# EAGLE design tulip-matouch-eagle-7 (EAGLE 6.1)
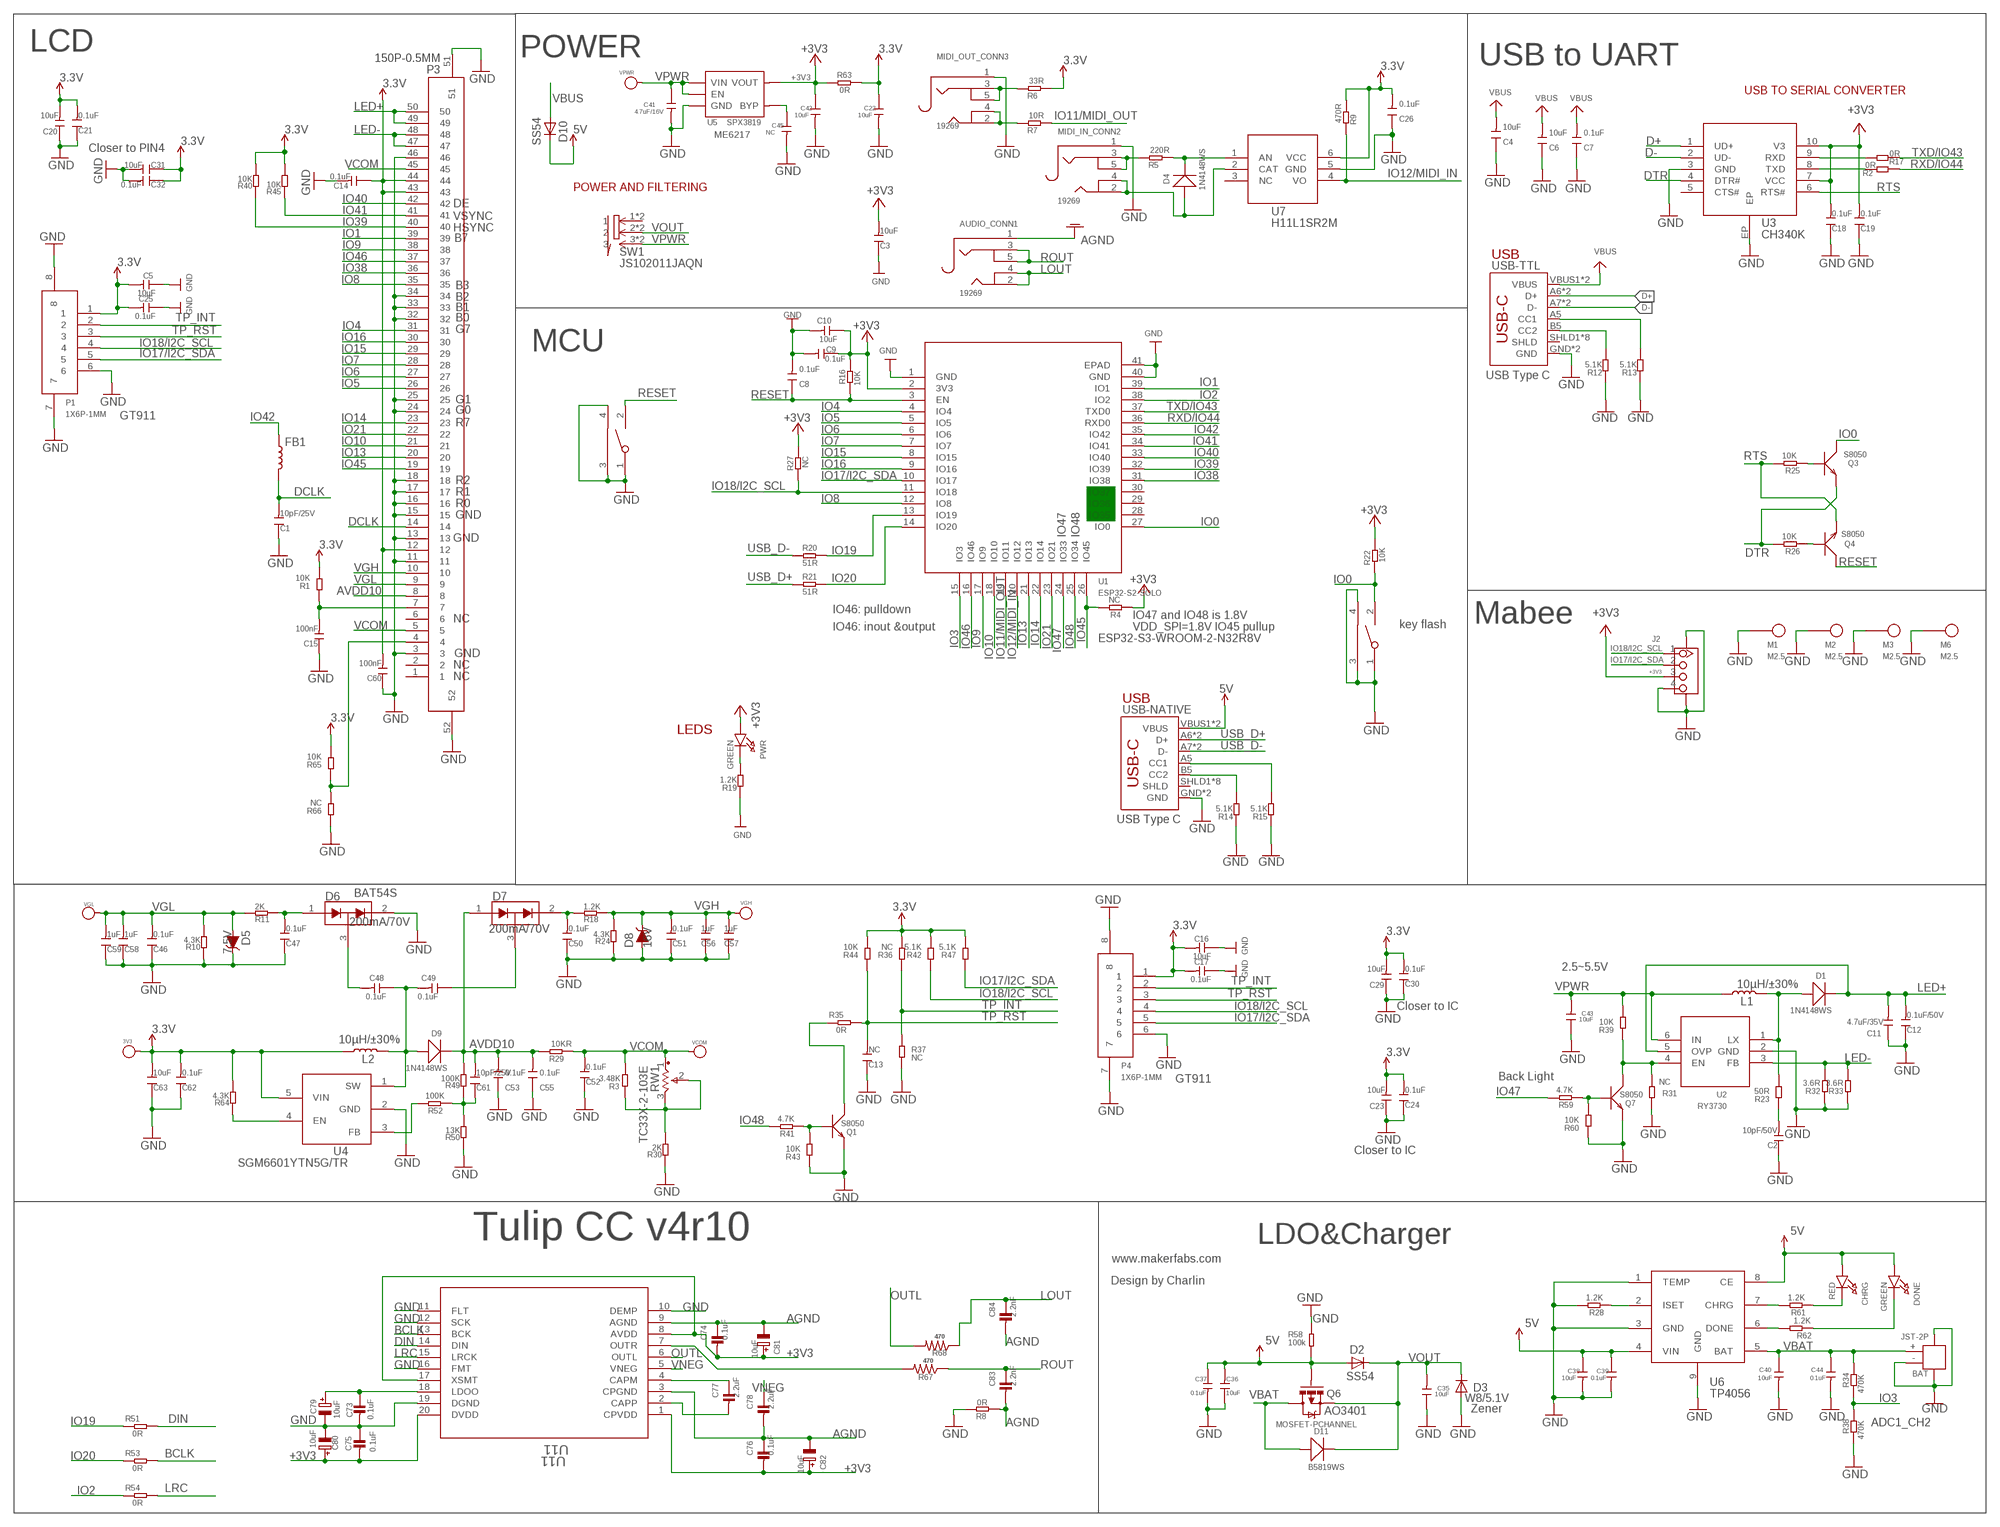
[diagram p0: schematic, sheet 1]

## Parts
3V3  PAD-TEST-POINT-CIRCLE'4545'  [TP_4545]
AUDIO_CONN1  19269  AUDIO_3.5MMJACK  [4UCONN_19269]
BAT  JST-2P  JST-2P-SMD'2.0'  [HW2-SMD-2.0-90D]
BOOT  TS24CA  [2*4*3.5MM]
C1  10pF/25V  DISCRETE_C-0603  [DISCRETE_C0603]
C2  10pF/50V  DISCRETE_C-0603  [DISCRETE_C0603]
C3  10uF  DISCRETE_C-0603  [DISCRETE_C0603]
C4  10uF  DISCRETE_C-0603  [DISCRETE_C0603]
C5  10uF  DISCRETE_C-0603  [DISCRETE_C0603]
C6  10uF  DISCRETE_C-0603  [DISCRETE_C0603]
C7  0.1uF  DISCRETE_C-0603  [DISCRETE_C0603]
C8  0.1uF  DISCRETE_C-0603  [DISCRETE_C0603]
C9  0.1uF  DISCRETE_C-0603  [DISCRETE_C0603]
C10  10uF  DISCRETE_C-0603  [DISCRETE_C0603]
C11  4.7uF/35V  DISCRETE_C-1206  [DISCRETE_C1206]
C12  0.1uF/50V  DISCRETE_C-0603  [DISCRETE_C0603]
C13  NC  DISCRETE_C-0603  [DISCRETE_C0603]
C14  0.1uF  DISCRETE_C-0603  [DISCRETE_C0603]
C15  100nF  DISCRETE_C-0603  [DISCRETE_C0603]
C16  10uF  DISCRETE_C-0603  [DISCRETE_C0603]
C17  0.1uF  DISCRETE_C-0603  [DISCRETE_C0603]
C18  0.1uF  DISCRETE_C-0603  [DISCRETE_C0603]
C19  0.1uF  DISCRETE_C-0603  [DISCRETE_C0603]
C20  10uF  DISCRETE_C-0603  [DISCRETE_C0603]
C21  0.1uF  DISCRETE_C-0603  [DISCRETE_C0603]
C22  10uF  C-0603  [0603]
C23  10uF  DISCRETE_C-0603  [DISCRETE_C0603]
C24  0.1uF  DISCRETE_C-0603  [DISCRETE_C0603]
C25  0.1uF  DISCRETE_C-0603  [DISCRETE_C0603]
C26  0.1uF  DISCRETE_C-0603  [DISCRETE_C0603]
C29  10uF  DISCRETE_C-0603  [DISCRETE_C0603]
C30  0.1uF  DISCRETE_C-0603  [DISCRETE_C0603]
C31  10uF  DISCRETE_C-0603  [DISCRETE_C0603]
C32  0.1uF  DISCRETE_C-0603  [DISCRETE_C0603]
C35  10uF  C-0603  [0603]
C36  10uF  C-0603  [0603]
C37  0.1uF  C-0603  [0603]
C38  10uF  C-0603  [0603]
C39  0.1uF  C-0603  [0603]
C40  10uF  C-0603  [0603]
C41  4.7uF/16V  C-0603  [0603]
C42  10uF  C-0603  [0603]
C43  10uF  C-0603  [0603]
C44  0.1uF  C-0603  [0603]
C45  NC  C-0603  [0603]
C46  0.1uF  DISCRETE_C-0603  [DISCRETE_C0603]
C47  0.1uF  DISCRETE_C-0603  [DISCRETE_C0603]
C48  0.1uF  DISCRETE_C-0603  [DISCRETE_C0603]
C49  0.1uF  DISCRETE_C-0603  [DISCRETE_C0603]
C50  0.1uF  DISCRETE_C-0603  [DISCRETE_C0603]
C51  0.1uF  DISCRETE_C-0603  [DISCRETE_C0603]
C52  0.1uF  DISCRETE_C-0603  [DISCRETE_C0603]
C53  0.1uF  DISCRETE_C-0603  [DISCRETE_C0603]
C55  0.1uF  DISCRETE_C-0603  [DISCRETE_C0603]
C56  1uF  DISCRETE_C-0603  [DISCRETE_C0603]
C57  1uF  DISCRETE_C-0603  [DISCRETE_C0603]
C58  1uF  DISCRETE_C-0603  [DISCRETE_C0603]
C59  1uF  DISCRETE_C-0603  [DISCRETE_C0603]
C60  100nF  DISCRETE_C-0603  [DISCRETE_C0603]
C61  10pF/25V  DISCRETE_C-0603  [DISCRETE_C0603]
C62  0.1uF  DISCRETE_C-0603  [DISCRETE_C0603]
C63  10uF  DISCRETE_C-0603  [DISCRETE_C0603]
C73  0.1uF  CAP_CERAMIC0805-NOOUTLINE  [0805-NO]
C74  0.1uF  CAP_CERAMIC0805-NOOUTLINE  [0805-NO]
C75  0.1uF  CAP_CERAMIC0805-NOOUTLINE  [0805-NO]
C76  0.1uF  CAP_CERAMIC0805-NOOUTLINE  [0805-NO]
C77  2.2uF  CAP_CERAMIC0805-NOOUTLINE  [0805-NO]
C78  2.2uF  CAP_CERAMIC0805-NOOUTLINE  [0805-NO]
C79  10uF  CAP_ELECTROLYTICPANASONIC_C  [PANASONIC_C]
C80  10uF  CAP_ELECTROLYTICPANASONIC_C  [PANASONIC_C]
C81  10uF  CAP_ELECTROLYTICPANASONIC_C  [PANASONIC_C]
C82  10uF  CAP_ELECTROLYTICPANASONIC_C  [PANASONIC_C]
C83  2.2nF  CAP_CERAMIC0805-NOOUTLINE  [0805-NO]
C84  2.2nF  CAP_CERAMIC0805-NOOUTLINE  [0805-NO]
CHRG  RED  LED0805_NOOUTLINE  [CHIPLED_0805_NOOUTLINE]
D1  1N4148WS  D'0805'  [SOD323]
D2  SS54  DIODE-DO-214AC  [DO-214AC]
D3  W8/5.1V  DIODE-SOD123  [SOD123]
D4  1N4148WS  D'0805'  [SOD323]
D5  7.5V  DIODE-ZENER-MMSZ5232BS  [SOD-323]
D6  200mA/70V  BAV99  [SOT23-3]
D7  200mA/70V  BAV99  [SOT23-3]
D8  16V  DIODE-ZENER-MMSZ5232BS  [SOD-323]
D9  1N4148WS  D'0805'  [SOD323]
D10  SS54  DIODE-DO-214AC  [DO-214AC]
D11  B5819WS  D'0805'  [SOD323]
DONE  GREEN  LED0805_NOOUTLINE  [CHIPLED_0805_NOOUTLINE]
FB1  INDUCTORFB-30OHM  [0603]
J2  GROVE-CONNECTOR-SMD'90D'  [HW4-SMD-2.0-90D]
L1  10µH/±30%  INDUCTOR-CR54-3.3UH  [CR54]
L2  10µH/±30%  INDUCTOR-CR54-3.3UH  [CR54]
M1  M2.5  [M2.5]
M2  M2.5  [M2.5]
M3  M2.5  [M2.5]
M6  M2.5  [M2.5]
MIDI_IN_CONN2  19269  AUDIO_3.5MMJACK  [4UCONN_19269]
MIDI_OUT_CONN3  19269  AUDIO_3.5MMJACK  [4UCONN_19269]
P1  1X6P-1MM  [1*6P-SMT1MM]
P3  150P-0.5MM  [1*50P-SMT0.5MM]
P4  1X6P-1MM  [1*6P-SMT1MM]
PWR  GREEN  LED0805_NOOUTLINE  [CHIPLED_0805_NOOUTLINE]
Q1  S8050  TRANSISTOR-NPN-SOT23  [SOT23]
Q3  S8050  TRANSISTOR-NPN-SOT23  [SOT23]
Q4  S8050  TRANSISTOR-NPN-SOT23  [SOT23]
Q6  MOSFET-PCHANNEL  [SOT23-3]
Q7  S8050  TRANSISTOR-NPN-SOT23  [SOT23]
R1  10K  DISCRETE_R-0603  [DISCRETE_R0603]
R2  0R  R-0603  [R0603]
R3  3.48K  DISCRETE_R-0603  [DISCRETE_R0603]
R4  NC  R-0603  [R0603]
R5  220R  R-0603  [R0603]
R6  33R  R-0603  [R0603]
R7  10R  R-0603  [R0603]
R8  0R  DISCRETE_R-0603  [DISCRETE_R0603]
R9  470R  R-0603  [R0603]
R10  4.3K  DISCRETE_R-0603  [DISCRETE_R0603]
R11  2K  DISCRETE_R-0603  [DISCRETE_R0603]
R12  5.1K  DISCRETE_R-0603  [DISCRETE_R0603]
R13  5.1K  DISCRETE_R-0603  [DISCRETE_R0603]
R14  5.1K  DISCRETE_R-0603  [DISCRETE_R0603]
R15  5.1K  DISCRETE_R-0603  [DISCRETE_R0603]
R16  10K  R-0603  [R0603]
R17  0R  R-0603  [R0603]
R18  1.2K  DISCRETE_R-0603  [DISCRETE_R0603]
R19  1.2K  DISCRETE_R-0603  [DISCRETE_R0603]
R20  51R  R-0603  [R0603]
R21  51R  R-0603  [R0603]
R22  10K  R-0603  [R0603]
R23  50R  DISCRETE_R-0603  [DISCRETE_R0603]
R24  4.3K  DISCRETE_R-0603  [DISCRETE_R0603]
R25  10K  R-0603  [R0603]
R26  10K  R-0603  [R0603]
R27  NC  R-0603  [R0603]
R28  1.2K  R-0603  [R0603]
R29  10KR  DISCRETE_R-0603  [DISCRETE_R0603]
R30  2K  DISCRETE_R-0603  [DISCRETE_R0603]
R31  NC  DISCRETE_R-0603  [DISCRETE_R0603]
R32  3.6R  DISCRETE_R-0603  [DISCRETE_R0603]
R33  3.6R  DISCRETE_R-0603  [DISCRETE_R0603]
R34  470K  R-0603  [R0603]
R35  0R  R-0603  [R0603]
R36  NC  DISCRETE_R-0603  [DISCRETE_R0603]
R37  NC  DISCRETE_R-0603  [DISCRETE_R0603]
R38  470K  R-0603  [R0603]
R39  10K  DISCRETE_R-0603  [DISCRETE_R0603]
R40  10K  DISCRETE_R-0603  [DISCRETE_R0603]
R41  4.7K  DISCRETE_R-0603  [DISCRETE_R0603]
R42  5.1K  DISCRETE_R-0603  [DISCRETE_R0603]
R43  10K  DISCRETE_R-0603  [DISCRETE_R0603]
R44  10K  DISCRETE_R-0603  [DISCRETE_R0603]
R45  10K  DISCRETE_R-0603  [DISCRETE_R0603]
R47  5.1K  DISCRETE_R-0603  [DISCRETE_R0603]
R49  100K  DISCRETE_R-0603  [DISCRETE_R0603]
R50  13K  DISCRETE_R-0603  [DISCRETE_R0603]
R51  0R  R-0603  [R0603]
R52  100K  DISCRETE_R-0603  [DISCRETE_R0603]
R53  0R  R-0603  [R0603]
R54  0R  R-0603  [R0603]
R58  100k  R-0603  [R0603]
R59  4.7K  DISCRETE_R-0603  [DISCRETE_R0603]
R60  10K  DISCRETE_R-0603  [DISCRETE_R0603]
R61  1.2K  R-0603  [R0603]
R62  1.2K  R-0603  [R0603]
R63  0R  R-0603  [R0603]
R64  4.3K  DISCRETE_R-0603  [DISCRETE_R0603]
R65  10K  DISCRETE_R-0603  [DISCRETE_R0603]
R66  NC  DISCRETE_R-0603  [DISCRETE_R0603]
R67  470  R-US_R0805  [R0805]
R68  470  R-US_R0805  [R0805]
RST  TS24CA  [2*4*3.5MM]
RW1  TC33X-2-103E  [TC33-3MM-SMD]
SW1  JS102011JAQN  [SMD-6-2.5MM]
U1  ESP32­S2­SOLO  [ESP32-­S2-­SOLO]
U2  RY3730  [SOT23-6]
U3  CH340K  [ESOP-10-EP-150MIL]
U4  SGM6601YTN5G/TR  [SOT-23-5]
U5  SPX3819  [SOT23-5]
U6  TP4056  [SOP8-1.27P]
U7  H11L1SR2M  [SOP-6-2.54MM]
U11  U11  PCM5101APW  [PW20_TEX]
USB-NATIVE  USB_C5  [USB-C-16P-5]
USB-TTL  USB_C5  [USB-C-16P-5]
VCOM  PAD-TEST-POINT-CIRCLE'4545'  [TP_4545]
VGH  PAD-TEST-POINT-CIRCLE'4545'  [TP_4545]
VGL  PAD-TEST-POINT-CIRCLE'4545'  [TP_4545]
VPWR  PAD-TEST-POINT-CIRCLE'4545'  [TP_4545]

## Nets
3.3V: 3V3.T C5.2 C14.1 C16.2 C17.2 C20.2 C21.2 C22.1 C23.2 C24.2 C25.2 C26.2 C29.2 C30.2 C31.1 C32.1 C60.2 C62.2 C63.2 L2.P$1 P1.1 P3.12 P3.43 P3.44 P4.1 R1.2 R6.1 R9.1 R36.2 R40.2 R42.2 R44.2 R45.2 R47.2 R63.2 R64.2 R65.2 U4.5(VIN) U7.6(VCC)
5V: C36.2 C37.1 C38.1 C39.1 CHRG.A D2.A D10.C DONE.A Q6.1(G) R58.1 U6.4(VIN) U6.8(CE) USB-NATIVE.VBUS1(VBUS) USB-NATIVE.VBUS2(VBUS)
+3V3: C3.2 C9.1 C10.1 C18.2 C19.2 C42.1 C74.2 C75.2 C76.2 C80.+ C81.+ C82.+ J2.3 PWR.A R4.1 R16.2 R22.2 R27.2 R63.1 U1.2(3V3) U3.7(VCC) U3.10(V3) U5.5(VOUT) U11.1(CPVDD) U11.8(AVDD) U11.17(XSMT) U11.20(DVDD)
AGND: AUDIO_CONN1.1 C74.1 C76.1 C78.2 C81.- C82.- C83.2 C84.2 R8.1 U11.3(CPGND) U11.9(AGND)
AVDD10: C53.2 C55.2 C61.2 D7.1(A1) D9.- P3.8 R29.2 R49.2
BCLK: R53.2 U11.13(BCK)
D+: U3.1(UD+) USB-TTL.A6(D+) USB-TTL.B6(D+)
D-: U3.2(UD-) USB-TTL.A7(D-) USB-TTL.B7(D-)
DCLK: C1.2 FB1.2 P3.14
DIN: R51.2 U11.14(DIN)
DTR: Q3.2(E) R26.2 U3.4(DTR#)
GND: BAT.3 BAT.4 BAT.- BOOT.1 BOOT.3 BOOT.4 C1.1 C2.1 C3.1 C4.1 C5.1 C6.1 C7.1 C8.2 C9.2 C10.2 C11.1 C12.1 C13.1 C14.2 C15.1 C16.1 C17.1 C18.1 C19.1 C20.1 C21.1 C22.2 C23.1 C24.1 C25.1 C26.1 C29.1 C30.1 C31.2 C32.2 C35.1 C36.1 C37.2 C38.2 C39.2 C40.2 C41.2 C42.2 C43.1 C44.2 C45.2 C46.1 C47.1 C50.1 C51.1 C52.1 C53.1 C55.1 C56.1 C57.1 C58.1 C59.1 C60.1 C62.1 C63.1 C73.2 C75.1 C79.- C80.- D3.A D5.C D6.2(C2) D8.A J2.4 J2.SS1 J2.SS2 M1.1 M2.1 M3.1 M6.1 MIDI_IN_CONN2.1 MIDI_OUT_CONN3.1 P1.6 P1.7 P1.8 P3.3 P3.11 P3.13 P3.15 P3.16 P3.17 P3.18 P3.24 P3.25 P3.32 P3.33 P3.34 P3.46 P3.51 P3.52 P4.6 P4.7 P4.8 Q1.2(E) Q7.2(E) R8.2 R10.1 R12.1 R13.1 R14.1 R15.1 R19.1 R24.1 R28.2 R30.1 R31.1 R32.1 R33.1 R37.2 R38.1 R43.1 R50.1 R58.2 R60.1 R66.1 RST.1 RST.3 RST.4 U1.1(GND) U1.40(GND) U1.41(EPAD) U2.2(GND) U3.3(GND) U3.EP U4.2(GND) U5.2(GND) U6.1(TEMP) U6.3(GND) U6.9(GND) U7.5(GND) U11.10(DEMP) U11.11(FLT) U11.12(SCK) U11.16(FMT) U11.19(DGND) USB-NATIVE.GND USB-NATIVE.GND2(GND) USB-TTL.GND USB-TTL.GND2(GND)
IO0: BOOT.2 Q3.3(C) R22.1 U1.27(IO0)
IO1: P3.39 U1.39(IO1)
IO2: R54.1 U1.38(IO2)
IO3: R34.1 R38.2 U1.15(IO3)
IO4: P3.31 U1.4(IO4)
IO5: P3.26 U1.5(IO5)
IO6: P3.27 U1.6(IO6)
IO7: P3.28 U1.7(IO7)
IO8: P3.35 U1.12(IO8)
IO9: P3.38 U1.17(IO9)
IO10: P3.21 U1.18(IO10)
IO11/MIDI_OUT: R7.1 U1.19(IO11)
IO12/MIDI_IN: R9.2 U1.20(IO12) U7.4(VO)
IO13: P3.20 U1.21(IO13)
IO14: P3.23 U1.22(IO14)
IO15: P3.29 U1.8(IO15)
IO16: P3.30 U1.9(IO16)
IO17/I2C_SDA: J2.2 P1.5 P4.5 R47.1 U1.10(IO17)
IO18/I2C_SCL: J2.1 P1.4 P4.4 R27.1 R42.1 U1.11(IO18)
IO19: R20.2 R51.1 U1.13(IO19)
IO20: R21.2 R53.1 U1.14(IO20)
IO21: P3.22 U1.23(IO21)
IO38: P3.36 U1.31(IO38)
IO39: P3.40 R40.1 U1.32(IO39)
IO40: P3.42 U1.33(IO40)
IO41: P3.41 R45.1 U1.34(IO41)
IO42: FB1.1 U1.35(IO42)
IO45: P3.19 R4.2 U1.26(IO45)
IO46: P3.37 U1.16(IO46)
IO47: R59.2 U1.24(IO33)
IO48: R41.2 U1.25(IO34)
LCD_RST: C15.2 P3.7 R1.1
LED+: C11.2 C12.2 D1.- P3.49 P3.50 U2.5(OVP)
LED-: P3.47 P3.48 R32.2 R33.2 U2.3(FB)
LOUT: AUDIO_CONN1.2 AUDIO_CONN1.4 C84.1 R68.1
LRC: R54.2 U11.15(LRCK)
N$1: C47.2 D6.1(A1) R11.1
N$2: Q4.1(B) R26.1
N$3: Q3.1(B) R25.1
N$4: C61.1 R49.1 R50.2 R52.1
N$5: P3.4 R65.1 R66.2
N$6: R15.2 USB-NATIVE.A5(CC1)
N$7: PWR.C R19.2
N$8: C48.2 D6.3(COM)
N$9: C48.1 C49.2 D9.+ L2.P$2 U4.1(SW)
N$10: R13.2 USB-TTL.A5(CC1)
N$11: R12.2 USB-TTL.B5(CC2)
N$12: C49.1 D7.3(COM)
N$13: C50.2 D7.2(C2) R18.2
N$14: R14.2 USB-NATIVE.B5(CC2)
N$15: R52.2 U4.3(FB)
N$16: R3.1 R30.2 RW1.2 RW1.3
N$17: D1.+ L1.P$2 R23.2 U2.1(LX)
N$18: Q1.3(C) R35.1
N$19: R64.1 U4.4(EN)
N$20: Q1.1(B) R41.1 R43.2
N$22: C2.2 R23.1
N$23: MIDI_IN_CONN2.3 MIDI_IN_CONN2.5 R5.2
N$24: Q7.3(C) R31.2 R39.1 U2.4(EN)
N$26: D4.- R5.1 U7.1(AN)
N$27: MIDI_OUT_CONN3.3 MIDI_OUT_CONN3.5 R6.2
N$29: Q7.1(B) R59.1 R60.2
N$30: R28.1 U6.2(ISET)
N$31: R61.2 U6.7(CHRG)
N$32: R62.2 U6.6(DONE)
N$33: CHRG.C R61.1
N$34: DONE.C R62.1
N$35: MIDI_OUT_CONN3.2 MIDI_OUT_CONN3.4 R7.2
N$36: D4.+ MIDI_IN_CONN2.2 MIDI_IN_CONN2.4 U7.2(CAT)
N$43: C73.1 C79.+ U11.18(LDOO)
N$44: R67.2 U11.7(OUTR)
N$45: C77.1 U11.4(CAPM)
N$46: R17.2 U3.9(RXD)
N$47: C77.2 U11.2(CAPP)
N$49: R2.2 U3.8(TXD)
N$76: C45.1 U5.4(BYP)
OUTL: R68.2 U11.6(OUTL)
RESET: C8.1 Q4.3(C) R16.1 RST.2 U1.3(EN)
ROUT: AUDIO_CONN1.3 AUDIO_CONN1.5 C83.1 R67.1
RTS: Q4.2(E) R25.2 U3.6(RTS#)
RXD/IO44: R2.1 U1.36(RXD0)
TP_INT: P1.2 P4.2 R36.1 R37.1
TP_RST: C13.2 P1.3 P4.3 R35.2 R44.1
TXD/IO43: R17.1 U1.37(TXD0)
USB_D+: R21.1 USB-NATIVE.A6(D+) USB-NATIVE.B6(D+)
USB_D-: R20.1 USB-NATIVE.A7(D-) USB-NATIVE.B7(D-)
VBAT: BAT.+ C40.1 C44.1 D11.+ Q6.3(D) R34.2 U6.5(BAT)
VBUS: C4.2 C6.2 C7.2 D10.A USB-TTL.VBUS1(VBUS) USB-TTL.VBUS2(VBUS)
VCOM: C52.2 P3.5 P3.45 R3.2 R29.1 RW1.1 VCOM.T
VGH: C51.2 C56.2 C57.2 D8.C P3.10 R18.1 R24.2 VGH.T
VGL: C46.2 C58.2 C59.2 D5.A P3.9 R10.2 R11.2 VGL.T
VNEG: C78.1 U11.5(VNEG)
VOUT: C35.2 D2.C D3.C D11.- Q6.2(S) SW1.2 SW1.2@1
VPWR: C41.1 C43.2 L1.P$1 R39.2 SW1.3 SW1.3@1 U2.6(IN) U5.1(VIN) U5.3(EN) VPWR.T
Unconnected: P3.1 P3.2 P3.6 SW1.1 SW1.1@1 U1.28(IO35) U1.29(IO36) U1.30(IO37) U3.5(CTS#) U7.3(NC) USB-NATIVE.SHLD1(SHLD) USB-NATIVE.SHLD2(SHLD) USB-NATIVE.SHLD3(SHLD) USB-NATIVE.SHLD4(SHLD) USB-NATIVE.SHLD5(SHLD) USB-NATIVE.SHLD6(SHLD) USB-NATIVE.SHLD7(SHLD) USB-NATIVE.SHLD8(SHLD) USB-TTL.SHLD1(SHLD) USB-TTL.SHLD2(SHLD) USB-TTL.SHLD3(SHLD) USB-TTL.SHLD4(SHLD) USB-TTL.SHLD5(SHLD) USB-TTL.SHLD6(SHLD) USB-TTL.SHLD7(SHLD) USB-TTL.SHLD8(SHLD)

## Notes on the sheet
- LCD | POWER
- USB to UART
- USB TO SERIAL CONVERTER
- ME6217
- Closer to PIN4
- POWER AND FILTERING
- DE
- VSYNC
- HSYNC
- B7
- USB
- B3
- B2
- B1
- B0
- G7
- MCU
- USB Type C
- G1
- G0
- GT911
- R7
- R2
- R1
- R0
- GND
- IO47 | IO48
- GND
- IO46: pulldown
- IO47 and IO48 is 1.8V
- NC | Mabee
- IO46: inout &output | VDD_SPI=1.8V IO45 pullup | key flash
- ESP32-S3-WROOM-2-N32R8V
- GND
- NC
- NC
- USB
- LEDS
- USB Type C
- BAT54S
- 2.5~5.5V
- Closer to IC
- GT911 | Back Light
- Closer to IC
- Tulip CC v4r10 | LDO&Charger
- www.makerfabs.com
- Design by Charlin
- AO3401 | Zener
- ADC1_CH2

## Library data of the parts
3V3 VCOM VGH VGL VPWR = Discrete:PAD-TEST-POINT-CIRCLE; PARTNO: DNP
AUDIO_CONN1 MIDI_IN_CONN2 MIDI_OUT_CONN3 = microbuilder:AUDIO_3.5MMJACK: 3.5MM Audio Jack These are normally connected as follows, from left-to right on the schematic symbol above: Tip: Left Audio Inner Ring: Right Audio Shell: Common/GND
BAT = Connector-new:JST-2P-SMD: 2P-SMD-1.0-90D:320110054;2P-SMD-2.0-90D:320110026
BOOT RST = sale:TS24CA
C1-C21 C23-C26 C29-C32 C46-C53 C55-C63 = A9G:DISCRETE_C*: Ceramic Capacitors
C22 C35-C45 = Discrete:C*: Ceramic Capacitors
C73-C78 C83 C84 = microbuilder:CAP_CERAMIC: Ceramic Capacitors
C79-C82 = microbuilder:CAP_ELECTROLYTIC: Electrolytic Capacitors
CHRG DONE PWR = microbuilder:LED: LED
D1 D4 D9 D11 = Discrete:D*
D2 D3 D10 = diode:DIODE-: DIODE
D5 D8 = SparkFun-DiscreteSemi:DIODE-ZENER: Zener Diode; PROD_ID: DIO-12442; VALUE: 5.6V
D6 D7 = SparkFun-DiscreteSemi:BAV99: Series-pair diode array Two small signal silicon diodes connected anode to cathode. Connections to all three nodes available. Link to datasheet SparkFun Products: SparkFun AutoDriver; PROD_ID: DIO-10647
FB1 = SparkFun-Coils:INDUCTOR: Inductors; PROD_ID: NDUC-07859
J2 = Connector-new:GROVE-CONNECTOR-SMD: 4P-SMD-2.0:320110030;4P-SMD-2.0-90D:320110032
L1 L2 = SparkFun-Coils:INDUCTOR: Inductors; PROD_ID: NDUC-11157; VALUE: 3.3µH/±30%/3.4A
M1-M3 M6 = sale:M2.5
P1 P4 = sale:1X6P-1MM
P3 = sale:1*50P-0.5MM
Q1 Q3 Q4 Q7 = Discrete:TRANSISTOR-NPN*: NPN audion
Q6 = User-Submitted:MOSFET-PCHANNEL: Generic PMOSFET IRLML2244 - TRANS-11153 (SOT-23 -20V -4.3A) (1.Gate 2.Source 3.Drain) FQP27P06 - COM-10349 (TO-220 -60V -27A) (1.Gate 2.Source 3.Drain); PROD_ID: TRANS-08285
R1 R3 R8 R10-R15 R18 R19 R23 R24 R29-R33 R36 R37 R39-R45 R47 R49 R50 R52 R59 R60 R64-R66 = A9G:DISCRETE_R*
R2 R4-R7 R9 R16 R17 R20-R22 R25-R28 R34 R35 R38 R51 R53 R54 R58 R61-R63 = Discrete:R*
R67 R68 = adafruit:R-US_: RESISTOR, American symbol
RW1 = sale:TC33X-2-103E
SW1 = sale:JS102011JAQN
U1 = self:ESP32­S2­SOLO
U2 = sale:RY3730
U3 = sale:CH340K
U4 = sale:SGM6601YTN5G/TR
U5 = IC:SPX3819
U6 = self:TP4056
U7 = sale:H11L1SR2M
U11 = pcm5101apw:PCM5101APW; COPYRIGHT: Copyright (C) 2022 Ultra Librarian. All rights reserved.; DIGI-KEY_PART_NUMBER_1: PCM5101APW-ND; MANUFACTURER_PART_NUMBER: PCM5101APW; MFR_NAME: Texas Instruments
USB-NATIVE USB-TTL = USBC:USB_C: USB Type C 16Pin Connector Super Speed pins not available on the 16-pin purely SMD connector so this part is best for USB 2.0 implementations. D1 and D2 are tied together enabling D+/- no matter which way the cable is plugged into the connector. The two channel configuration pins (CC1/2) are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

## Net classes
0 default: width 0.203 mm
1 vbat: width 0.254 mm, drill 0.305 mm, clearance 0.152 mm

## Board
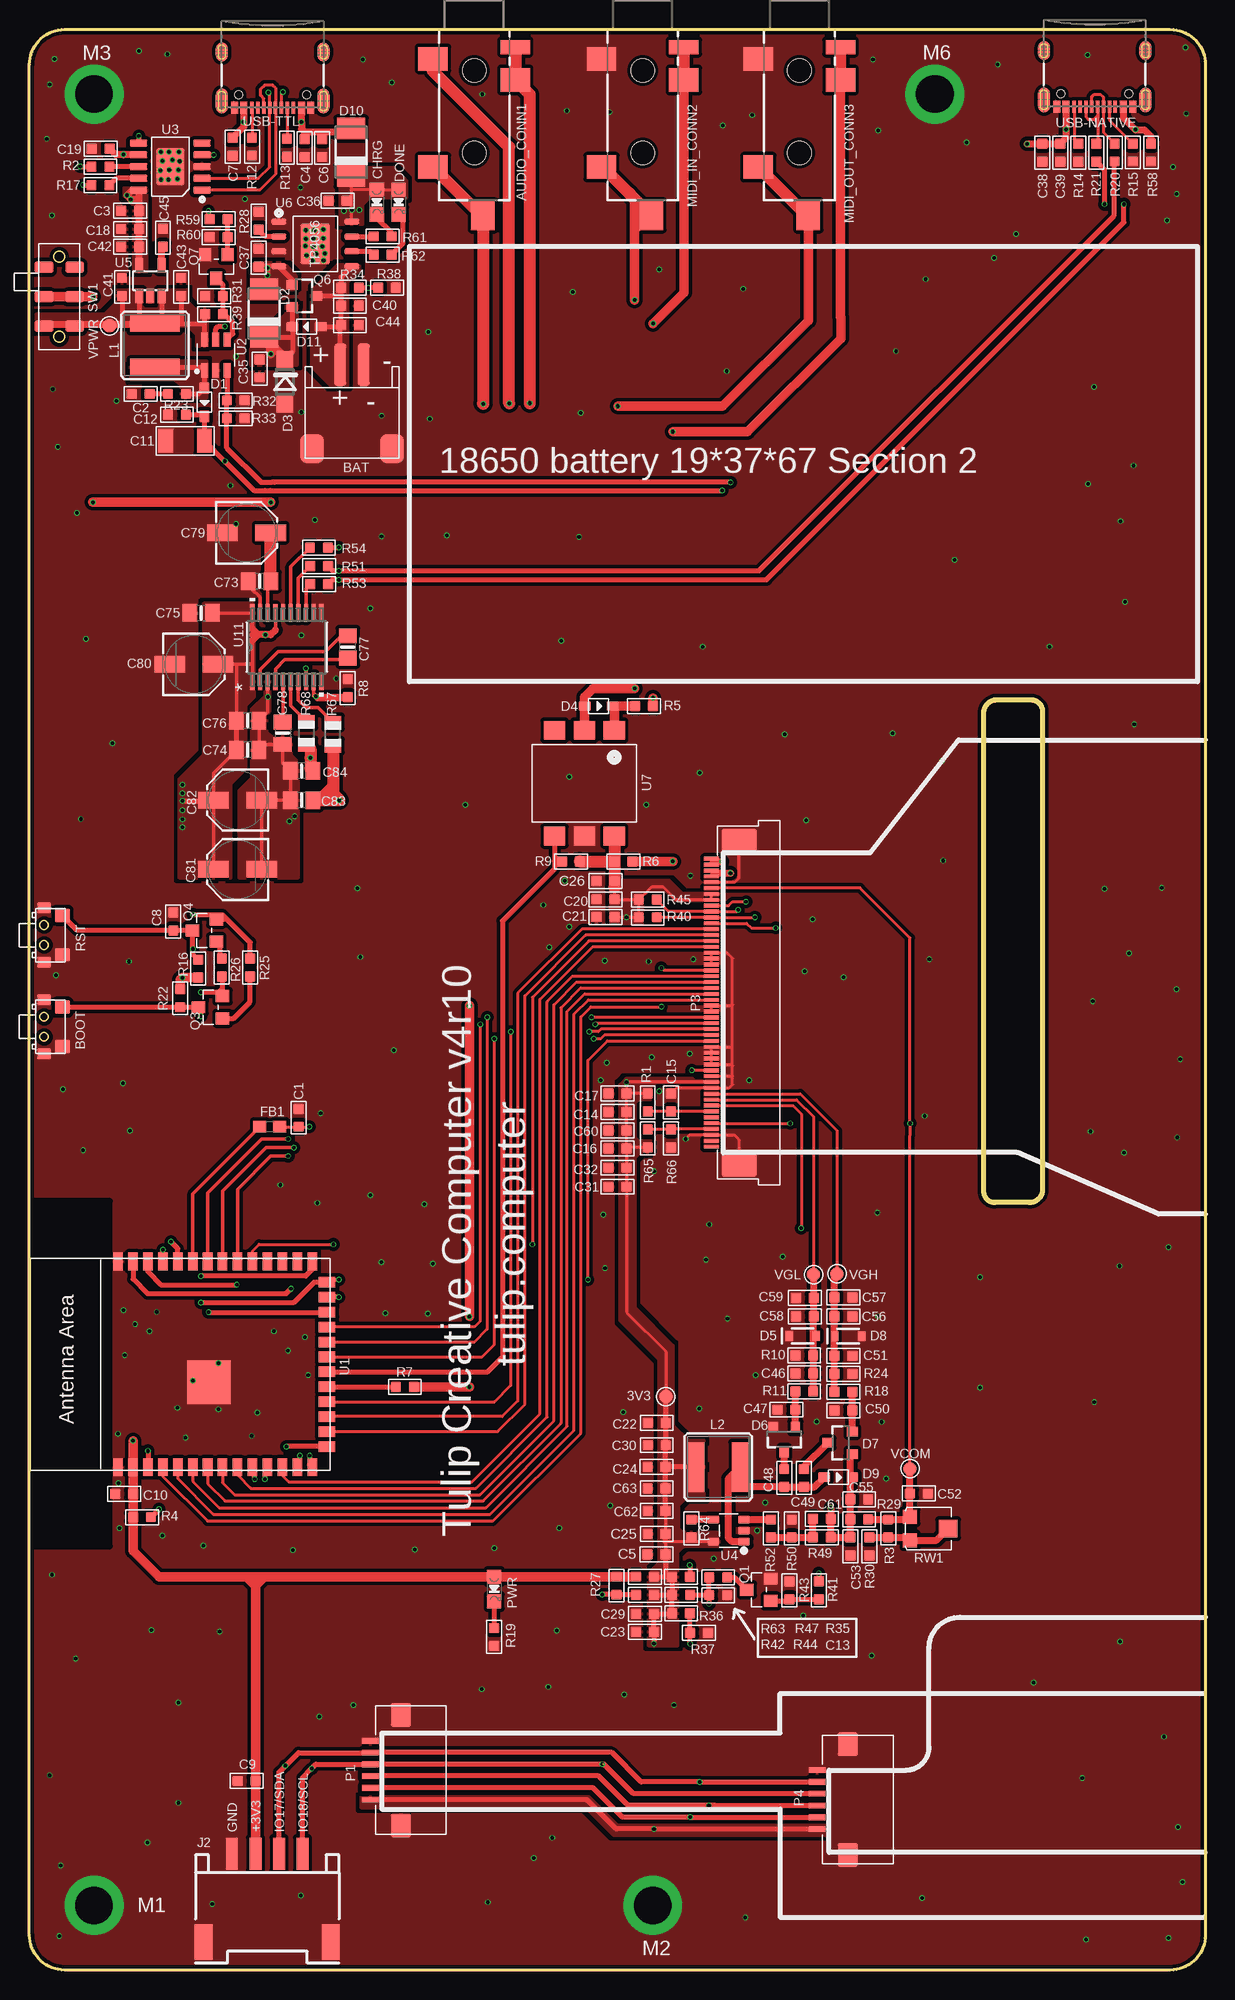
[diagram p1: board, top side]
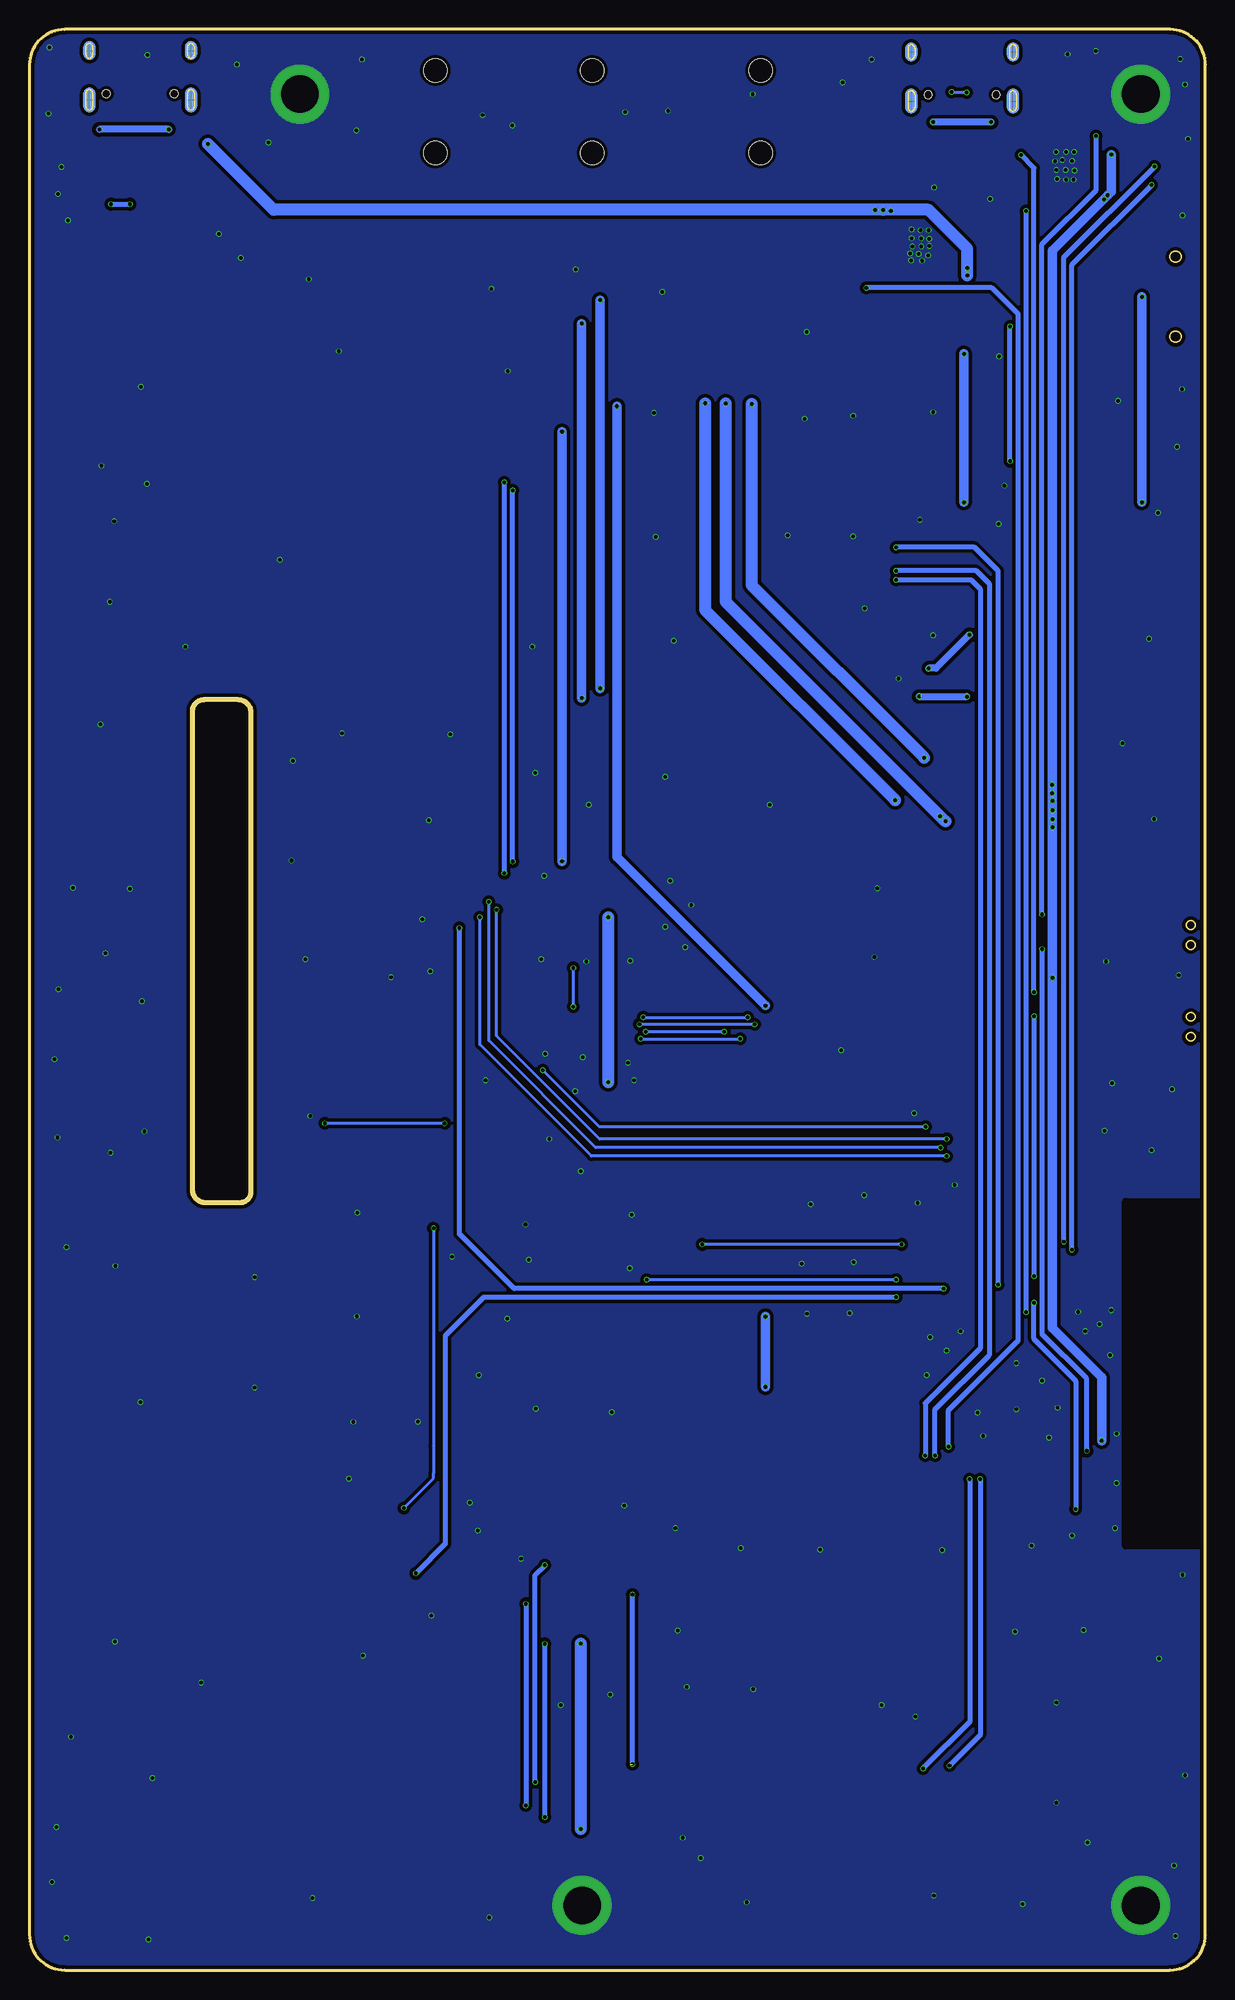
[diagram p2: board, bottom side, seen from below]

Size 100 x 165 mm. Coordinates in mm from the lower left corner, seen from the top.
Outline: 100,162 100,3 arc-90 97,0 3,0 arc-90 0,3 0,162 arc-90 3,165 97,165 arc-90 100,162
Outline: 85.03,65.25 82.09,65.25 arc-90 81.15,66.19 81.15,106.91 arc-90 82.25,108 85.17,108 arc-90 86.15,107.01 86.15,66.38 arc-90 85.03,65.25
Copper layers (1*16): Top 0.035mm / dielectric 1.5mm / Bottom 0.035mm
Design rules: minimum track width 6mil, minimum drill 10mil, track to track 6mil, track to pad 6mil, pad to pad 6mil, via to via 6mil, smd to smd 0mil, copper to edge 10mil, drill to drill 10mil, minimum pad ring 3mil, minimum via ring 3mil, stop-mask expansion 2mil, vias tented up to drill 100mil, thermal gap 0mil
tRestrict: area 0,36.1 to 6.8,65.4; area -3.4,136 to -2.6,142.5
bRestrict: area 0,36.1 to 6.8,65.4

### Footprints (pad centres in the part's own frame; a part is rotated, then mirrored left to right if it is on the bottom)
TP_4545 = smd 1.143 x 1.143: T 0,0
4UCONN_19269 = smd 2 x 2.5: 1 2.5,-3.5; 2 11.7,-3.5; 3 4.3,3.5 | smd 2.5 x 2: 4 15.8,0.75 | smd 1.2 x 2.5: 5 1.5,3.5 | hole 2: 3.5,0; 10.5,0
HW2-SMD-2.0-90D = smd 2 x 2.4: 3 3.4,-2.181; 4 -3.4,-2.181 | smd 1 x 3.6: + -1,4.953; - 1,4.953
2*4*3.5MM = smd 1.15 x 1.3: 1 -1.675,0; 2 1.675,0 | smd 0.9 x 1.2: 3 2.3,1.55; 4 -2.3,1.55
DISCRETE_C0603 = smd 0.889 x 0.889: 1 -0.762,0; 2 0.762,0
DISCRETE_C1206 = smd 1.27 x 2.032: 1 -1.651,0; 2 1.651,0
0603 = smd 0.889 x 0.889: 1 -0.762,0; 2 0.762,0
0805-NO = smd 1.24 x 1.5: 1 -0.95,0; 2 0.95,0
PANASONIC_C = smd 2.6 x 1.4: + 2.05,0; - -2.05,0
CHIPLED_0805_NOOUTLINE = smd 1.2 x 1.2: A 0,-1.05; C 0,1.05
SOD323 = smd 1 x 0.8: + -1.2,0; - 1.2,0
DO-214AC = smd 1.8 x 2.4: A 2.025,0; C -2.025,0
SOD123 = smd 1.4 x 1.4: A 1.9,0; C -1.9,0
SOD-323 = smd 0.63 x 0.83: A 1.15,0; C -1.15,0
SOT23-3 = smd 0.8 x 0.9: 1 -0.95,-1; 2 0.95,-1; 3 0,1.1
0603' = smd 1.1 x 1: 1 -0.85,0; 2 0.85,0
HW4-SMD-2.0-90D = smd 1.01 x 2.74: 1 -3,-0.1; 2 -1,-0.1; 3 1,-0.1; 4 3,-0.1 | smd 1.5 x 3: SS1 -5.4,7.4; SS2 5.4,7.4
CR54 = smd 4.2 x 1.4: P$1 0,1.85; P$2 0,-1.85
M2.5 = drill 3.2 pad 5: 1 0,0
1*6P-SMT1MM = smd 0.5 x 1.5: 1 -2.5,0; 2 -1.5,0; 3 -0.5,0; 4 0.5,0; 5 1.5,0; 6 2.5,0 | smd 2 x 1.7: 7 4.7,-2.6; 8 -4.7,-2.6
1*50P-SMT0.5MM = smd 0.3 x 1.3: 1 -12.25,0; 2 -11.75,0; 3 -11.25,0; 4 -10.75,0; 5 -10.25,0; 6 -9.75,0; 7 -9.25,0; 8 -8.75,0; 9 -8.25,0; 10 -7.75,0; 11 -7.25,0; 12 -6.75,0; 13 -6.25,0; 14 -5.75,0; 15 -5.25,0; 16 -4.75,0; 17 -4.25,0; 18 -3.75,0; 19 -3.25,0; 20 -2.75,0; 21 -2.25,0; 22 -1.75,0; 23 -1.25,0; 24 -0.75,0; 25 -0.25,0; 26 0.25,0; 27 0.75,0; 28 1.25,0; 29 1.75,0; 30 2.25,0; 31 2.75,0; 32 3.25,0; 33 3.75,0; 34 4.25,0; 35 4.75,0; 36 5.25,0; 37 5.75,0; 38 6.25,0; 39 6.75,0; 40 7.25,0; 41 7.75,0; 42 8.25,0; 43 8.75,0; 44 9.25,0; 45 9.75,0; 46 10.25,0; 47 10.75,0; 48 11.25,0; 49 11.75,0; 50 12.25,0 | smd 2 x 3: 51 13.79,-2.35; 52 -13.79,-2.35
SOT23 = smd 1.016 x 1.143: 1 -0.95,-1.016; 2 0.95,-1.016; 3 0,1.016
DISCRETE_R0603 = smd 0.889 x 0.889: 1 -0.762,0; 2 0.762,0
R0603 = smd 0.889 x 0.889: 1 -0.762,0; 2 0.762,0
R0805 = smd 1.1 x 1.4: 1 -1,0; 2 1,0
TC33-3MM-SMD = smd 1.2 x 1.2: 1 -1,-1.625; 2 1,-1.625 | smd 1.5 x 1.6: 3 0,1.625
SMD-6-2.5MM = smd 1 x 1.6: 1 -2.5,1.3; 1@1 -2.5,-1.3; 2 0,1.3; 2@1 0,-1.3; 3 2.5,1.3; 3@1 2.5,-1.3
ESP32-­S2-­SOLO = smd 1.5 x 0.9: 1 -8.75,5.26; 2 -8.75,3.99; 3 -8.75,2.72; 4 -8.75,1.45; 5 -8.75,0.18; 6 -8.75,-1.09; 7 -8.75,-2.36; 8 -8.75,-3.63; 9 -8.75,-4.9; 10 -8.75,-6.17; 11 -8.75,-7.44; 12 -8.75,-8.71; 13 -8.75,-9.98; 14 -8.75,-11.25; 27 8.75,-11.25; 28 8.75,-9.98; 29 8.75,-8.71; 30 8.75,-7.44; 31 8.75,-6.17; 32 8.75,-4.9; 33 8.75,-3.63; 34 8.75,-2.36; 35 8.75,-1.09; 36 8.75,0.18; 37 8.75,1.45; 38 8.75,2.72; 39 8.75,3.99; 40 8.75,5.26 | smd 0.9 x 1.5: 15 -6.985,-12.5; 16 -5.715,-12.5; 17 -4.445,-12.5; 18 -3.175,-12.5; 19 -1.905,-12.5; 20 -0.635,-12.5; 21 0.635,-12.5; 22 1.905,-12.5; 23 3.175,-12.5; 24 4.445,-12.5; 25 5.715,-12.5; 26 6.985,-12.5 | smd 3.7 x 3.7: 41 -1.5,-2.46
SOT23-6 = smd 1.2 x 0.6: 1 -1.3,0.95; 2 -1.3,0; 3 -1.3,-0.95; 4 1.3,-0.95; 5 1.3,0; 6 1.3,0.95
ESOP-10-EP-150MIL = smd 1.5 x 0.6: 1 -2.7,2; 2 -2.7,1; 3 -2.7,0; 4 -2.7,-1; 5 -2.7,-2; 6 2.7,-2; 7 2.7,-1; 8 2.7,0; 9 2.7,1; 10 2.7,2 | smd 2.4 x 3.2: EP 0,0
SOT-23-5 = smd 0.7 x 1: 1 -0.95,-1.3; 2 0,-1.3; 3 0.95,-1.3; 4 0.95,1.3; 5 -0.95,1.3
SOT23-5 = smd 0.69 x 1.2: 1 -0.95,-1.3; 2 0,-1.3; 3 0.95,-1.3; 4 0.95,1.3; 5 -0.95,1.3
SOP8-1.27P = smd 1.27 x 0.51: 1 -3.1,1.905; 2 -3.1,0.635; 3 -3.1,-0.635; 4 -3.1,-1.905; 5 3.1,-1.905; 6 3.1,-0.635; 7 3.1,0.635; 8 3.1,1.905 | smd 2.5 x 3.4: 9 0,0
SOP-6-2.54MM = smd 1.6 x 1.8: 1 -4.5,2.54; 2 -4.5,0; 3 -4.5,-2.54; 4 4.5,-2.54; 5 4.5,0; 6 4.5,2.54
PW20_TEX = smd 1.473 x 0.356: 1 -2.921,2.925; 2 -2.921,2.275; 3 -2.921,1.625; 4 -2.921,0.975; 5 -2.921,0.325; 6 -2.921,-0.325; 7 -2.921,-0.975; 8 -2.921,-1.625; 9 -2.921,-2.275; 10 -2.921,-2.925; 11 2.921,-2.925; 12 2.921,-2.275; 13 2.921,-1.625; 14 2.921,-0.975; 15 2.921,-0.325; 16 2.921,0.325; 17 2.921,0.975; 18 2.921,1.625; 19 2.921,2.275; 20 2.921,2.925
USB-C-16P-5 = smd 0.3 x 1: A5 -1.25,-0.34; A6 -0.25,-0.34; A7 0.25,-0.34; A8 1.25,-0.34; B5 1.75,-0.34; B6 0.75,-0.34; B7 -0.75,-0.34; B8 -1.75,-0.34 | smd 0.6 x 1: GND -3.225,-0.34; GND2 3.225,-0.34; VBUS1 -2.45,-0.34; VBUS2 2.45,-0.34 | smd 1 x 2.1: SHLD1 -4.32,-0.915; SHLD2 4.32,-0.915 | smd 1 x 2.1 bottom: SHLD3 -4.32,-0.915; SHLD4 4.32,-0.915 | smd 1 x 1.6: SHLD5 -4.32,-5.095; SHLD8 4.32,-5.095 | smd 1 x 1.6 bottom: SHLD6 -4.32,-5.095; SHLD7 4.32,-5.095 | hole 0.65: -2.89,-1.445; 2.89,-1.445

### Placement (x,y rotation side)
3V3  54.13,48.77 270 top
AUDIO_CONN1  37.82,165 270 top
BAT  27.43,131.53 0 top
BOOT  2.8,80.2 90 top
C1  22.89,72.47 270 top
C2  9.47,134.01 0 top
C3  8.56,149.58 0 top
C4  23.39,154.91 90 top
C5  53.31,35.36 0 top
C6  24.89,154.91 90 top
C7  17.3,155.02 90 top
C8  12.24,89.15 90 top
C9  18.47,16.08 180 top
C10  8.05,40.49 180 top
C11  13.23,130.02 0 top
C12  12.55,132.23 0 top
C13  58.57,31.88 180 top
C14  50.01,72.95 180 top
C15  54.56,73.76 270 top
C16  50.01,69.85 0 top
C17  50.01,74.52 0 top
C18  8.56,148.03 0 top
C19  6.07,154.86 0 top
C20  48.99,91.04 0 top
C21  49,89.54 0 top
C22  53.35,46.52 180 top
C23  52.34,28.76 0 top
C24  53.34,42.77 0 top
C25  53.34,37.08 0 top
C26  49,92.58 0 top
C29  52.35,30.3 0 top
C30  53.35,44.63 0 top
C31  50.01,66.61 180 top
C32  50.01,68.22 180 top
C35  19.58,136.17 90 top
C36  26.21,150.44 0 top
C37  19.51,145.59 90 top
C38  86.13,154.51 270 top
C39  87.66,154.51 270 top
C40  27.25,141.5 0 top
C41  7.87,143.1 90 top
C42  8.56,146.53 180 top
C43  12.9,143.1 270 top
C44  27.25,139.85 0 top
C45  11.35,147.29 90 top
C46  65.89,50.72 0 top
C47  64.36,47.65 0 top
C48  64.19,41.83 90 top
C49  65.86,41.83 270 top
C50  69.22,47.57 0 top
C51  69.22,52.22 180 top
C52  75.64,40.51 180 top
C53  69.8,36.02 90 top
C55  70.56,40.03 180 top
C56  69.22,55.58 180 top
C57  69.22,57.2 180 top
C58  65.94,55.58 0 top
C59  65.94,57.15 0 top
C60  50.01,71.37 0 top
C61  67.39,38.35 0 top
C62  53.34,39.04 0 top
C63  53.34,40.97 0 top
C73  19.58,118.08 180 top
C74  18.57,103.73 180 top
C75  14.6,115.39 0 top
C76  18.57,106.22 180 top
C77  27.08,112.5 90 top
C78  21.54,105.16 270 top
C79  18.47,122.2 0 top
C80  14,111.02 0 top
C81  17.7,93.57 180 top
C82  17.7,99.47 180 top
C83  23.16,99.47 180 top
C84  23.16,101.96 180 top
CHRG  29.54,150.32 180 top
D1  14.88,133.3 270 top
D2  19.96,140.87 90 top
D3  21.72,135.03 270 top
D4  48.41,107.47 0 top
D5  65.76,53.92 0 top
D6  64.19,45.16 180 top
D7  68.99,44.83 90 top
D8  69.62,53.9 0 top
D9  68.78,41.91 0 top
D10  27.36,154.56 90 top
D11  23.57,139.73 180 top
DONE  31.39,150.32 180 top
FB1  [0603']  20.45,71.7 0 top
J2  20.22,9.79 180 top
L1  10.67,138.15 0 top
L2  58.57,42.77 90 top
M1  5.5,5.5 0 top
M2  53,5.5 0 top
M3  5.5,159.5 0 top
M6  77,159.5 0 top
MIDI_IN_CONN2  52.15,165 270 top
MIDI_OUT_CONN3  65.48,165 270 top
P1  29,17 90 top
P3  58,82.25 90 top
P4  67,14.5 90 top
PWR  39.52,32.4 180 top
Q1  62.03,32.33 90 top
Q3  15.41,81.86 90 top
Q4  14.88,88.39 90 top
Q6  23.34,142.34 270 top
Q7  15.9,144.83 180 top
R1  52.58,73.76 90 top
R2  6.05,153.34 0 top
R3  73.03,37.54 90 top
R4  9.58,38.51 0 top
R5  52.27,107.47 0 top
R6  50.52,94.26 0 top
R7  31.93,49.58 0 top
R8  27.08,108.99 90 top
R9  46.05,94.26 180 top
R10  65.89,52.27 0 top
R11  65.89,49.2 0 top
R12  18.92,155.04 90 top
R13  21.89,154.94 90 top
R14  89.2,154.51 90 top
R15  93.83,154.53 90 top
R16  14.35,85.14 270 top
R17  6.05,151.76 0 top
R18  69.22,49.15 0 top
R19  39.52,28.32 90 top
R20  92.28,154.53 270 top
R21  90.73,154.51 270 top
R22  12.83,82.63 90 top
R23  12.55,134.01 0 top
R24  69.22,50.7 180 top
R25  18.77,85.24 90 top
R26  16.37,85.24 270 top
R27  49.91,32.69 90 top
R28  19.48,148.74 90 top
R29  70.56,38.33 180 top
R30  71.42,36.02 90 top
R31  15.7,142.32 0 top
R32  17.55,133.45 180 top
R33  17.55,131.93 180 top
R34  27.25,143.03 180 top
R35  58.57,33.4 180 top
R36  55.42,30.33 180 top
R37  56.95,28.68 0 top
R38  30.4,143.03 180 top
R39  15.7,140.79 180 top
R40  52.58,89.51 180 top
R41  67.13,32.28 90 top
R42  52.35,31.91 0 top
R43  64.64,32.28 270 top
R44  55.43,31.9 180 top
R45  52.58,91.01 180 top
R47  55.41,33.43 180 top
R49  67.39,36.78 0 top
R50  64.82,37.54 270 top
R51  24.64,119.35 180 top
R52  63.07,37.54 90 top
R53  24.64,117.83 180 top
R54  24.61,120.95 180 top
R58  95.38,154.53 270 top
R59  16.1,148.87 180 top
R60  16.1,147.35 0 top
R61  30.02,147.4 180 top
R62  30.05,145.85 180 top
R63  52.35,33.45 0 top
R64  56.29,37.54 270 top
R65  52.58,70.71 270 top
R66  54.56,70.71 90 top
R67  25.81,105.08 90 top
R68  23.57,105.16 90 top
RST  2.8,88 90 top
RW1  76.5,37.54 270 top
SW1  2.54,142.27 270 top
U1  12.8,51.5 90 top
U2  15.85,137.31 90 top
U3  11.99,153.34 180 top
U4  59.46,37.36 90 top
U5  10.29,143.64 0 top
U6  24.31,146.76 0 top
U7  47.19,100.91 270 top
U11  21.89,112.47 90 top
USB-NATIVE  90.58,158.1 180 top
USB-TTL  20.69,157.99 180 top
VCOM  74.88,42.62 0 top
VGH  68.68,59.21 0 top
VGL  66.67,59.13 90 top
VPWR  6.81,139.8 0 top

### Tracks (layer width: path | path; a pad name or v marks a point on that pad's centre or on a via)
3.3V  (via drill 0.3)
  Top 0.254: C16.2 C60.2 C14.1 C17.2 | R65.2 50.77,69.95 C16.2 | R1.2 C17.2 | C17.2 v50.77,75.5 P3.12 | R45.2 52.91,92.1 53.9,92.1 55,91 P3.43 P3.44 | R45.2 R40.2 51.79,89.54 C21.2 | C20.2 51.79,91.04 R45.2 | C16.2 C32.1 C31.1 50.78,55.93 54.11,52.59 C22.1 54.08,46.49 54.08,36.41 | 54.08,36.41 C5.2 | U4.5 56.31,36.41 | 56.31,36.41 54.08,36.41 | R64.2 56.31,36.78 56.31,36.41 | R6.1 49.76,95.68 49.73,95.71
  Top 0.305: C20.2 49.76,92.05 C26.2
  Top 0.406: P4.1 v53.11,12 49.9,12 47.4,14.5 P1.1 | R44.2 R36.2 54.63,30.3 C29.2 C23.2 v53.11,27.77 v53.11,27.76 | R42.2 54.65,31.91 R44.2 | R44.2 54.66,33.41 R47.2 54.62,33.45 54.05,33.45 | R63.2 54.05,33.45 | C5.2 54.08,33.48 54.05,33.45 | L2.P$1 C24.2 | 54.08,36.41 54.08,37.06 C25.2 | C62.2 C63.2 C24.2 | C24.2 C30.2 C22.1 54.11,48.75 3V3.T
  Top 1.016: R9.1 R6.1 | U7.6 49.73,95.71 49.73,92.07 49.76,92.05
  Bottom 1.016: v50.77,75.5 v50.77,89.5 | v53.11,12 v53.11,27.76
  pour Top: 28.22,14.76 47.6,14.76 50.01,12.34 67.74,12.34 67.74,11.43 49.68,11.43 47.35,13.77 28.22,13.77
  pour Top: 52.65,27.53 52.65,33.78 53.54,34.67 53.54,51.87 50.22,55.19 50.22,75.31 50.67,75.77 50.77,75.87 56.36,75.87 56.59,75.64 58.6,75.64 58.6,75.41 53.26,75.41 52.88,75.03 52.88,73.99 51.79,73.99 51.49,73.69 51.49,70.84 51.79,70.54 52.86,70.54 52.86,69.44 51.92,69.44 51.49,69.01 51.49,56.36 54.74,53.11 54.74,46.35 56.03,45.06 57.38,45.06 57.38,40.08 55.8,40.08 55.19,39.47 55.19,37.59 55.52,37.26 58.62,37.26 58.62,35.97 55.63,35.97 55.12,35.46 55.12,27.64 55.12,27.53
  pour Top: 49.35,89 52.2,89 52.2,91.29 52.78,91.87 53.98,91.87 54.89,90.96 58.65,90.96 58.65,91.54 55.58,91.54 54.66,92.46 54.48,92.63 50.04,92.63 49.35,91.95
5V  (via drill 0.3)
  Top 0.254: U6.8 27.41,150.42 | 27.41,150.42 27.41,151.33 | 27.41,151.33 27.41,152.48 D10.C | C36.2 27.38,150.44 27.41,150.42 | 27.41,151.33 27.44,151.37 CHRG.A DONE.A
  Top 0.406: 19.53,144.86 U6.4 22.34,143.72 Q6.1 | 19.53,144.86 C37.1 | v27.41,149.66 | D2.A 20.24,143.17 v20.24,144.09 v20.24,144.73 19.66,144.73 19.53,144.86
  Top 0.61: USB-NATIVE.VBUS1 93.03,157.49 94.06,156.46 94.11,156.46 | v88.14,156.5 88.13,157.08 USB-NATIVE.VBUS2 88.13,155.75 C39.1 C38.1 v84.84,155.27 | 94.11,156.46 94.82,156.46 95.38,155.91 R58.1 | v94.06,156.49 94.08,156.49 94.11,156.46
  Bottom 0.61: v88.14,156.5 94.05,156.5 v94.06,156.49
  Bottom 1.016: v84.84,155.27 79.22,149.66 v27.41,149.66 23.55,149.66 20.24,146.35 v20.24,144.09
  other vias: 28.07,149.66 26.75,149.58
  pour Top: 26.42,148.41 26.42,153.29 30.96,153.29 32.05,152.2 32.05,150.65 28.93,150.65 28.35,150.06 28.35,148.51 28.35,148.41
  pour Top: 22.58,142.93 18.97,142.93 18.97,144.75 18.97,145.11 21.51,145.11 22.58,144.04
+3V3  (via drill 0.3)
  Top 0.305: 18.97,113.56 U11.20 C75.2 | 18.97,113.56 18.97,110.9 | U11.1 | U11.17 20.92,113.94 | 19,113.54 18.97,113.56 | C80.+ 17.7,111.02 | 17.7,111.02 18.84,111.02 18.97,110.9 | C76.2 17.62,110.94 17.7,111.02 | C74.2 15.65,101.77 C82.+ C81.+ | U11.8 v23.52,110.69 | v23.52,110.69 | U11.1 18.97,110.9 | 18.97,110.9
  Top 0.406: 8.02,154.34 v8,154.36 | C74.2 C76.2 | v13,99.4 15.59,99.4 C82.+
  Top 0.61: 20.92,113.94 20.52,113.54 v20.06,113.54 19.43,113.54 | 19.43,113.54 19,113.54 | U3.7 8.02,154.34 7.36,154.34 C19.2 | v8.31,150.9 8.74,151.34 U3.10 9.32,151.31 9.32,150.44 | 18.85,114.22 18.85,114.12 19.43,113.54 | 19.43,113.54 18.82,112.93 | U5.5 9.34,146.52 C42.1 C18.2 C3.2 9.32,150.44 | v8.61,150.55 9.22,150.55 9.32,150.44
  Top 0.813: 19.48,33.45 11.04,33.45 11.02,33.43 8.81,35.64 R4.1 C10.1 U1.2 v8.81,45 | 19.48,33.45 PWR.A R27.2 R63.1 | J2.3 C9.1 19.23,32.69 | 19.23,32.69 19.23,33.19 19.48,33.45 | R22.2 12.83,84.21 v13,84.38 R16.2 | 19.23,32.69 19.99,33.45 | 19.23,32.69 19.18,32.69 18.47,33.4
  Bottom 0.61: v20.06,113.54 22.91,110.69 v23.52,110.69
  Bottom 0.813: v8.81,45 8.81,50.39 13,54.58 v13,84.38 v13,99.4 13,146.21 v8.31,150.9 8,151.21 v8,154.36
  other vias: 13.03,100.77 13,97.83 13.03,100.06 13,98.61 13,97.16
  pour Top: 15.44,116.26 19.1,116.26 19.1,108.18 18.39,107.47 18.39,102.08 17.12,100.81 17.12,92.81 12.75,92.81 12.75,101.3 14.83,103.38 14.83,116.26
  pour Top: 8.86,144.35 8.86,149.99 8.05,150.8 8.05,151.56 9.96,151.56 9.96,144.4 9.96,144.35
AGND  (via drill 0.3)  (1 unrouted)
  Top 0.254: R8.1 24.49,108.23 24.17,108.55 U11.9 24.17,108.29 v24.35,108.28
  Top 0.305: C81.- C82.- C83.2 C84.2 21.54,102.63 C78.2 19.63,104.21 19.52,104.32 | C74.1 19.52,104.32 | 19.52,104.32 C76.1 20.27,106.97 v20.27,108.25 U11.3 | 24.18,108.84 24.18,108.31 24.49,108 27.15,108 27.15,108.43 27.03,108.43 26.95,108.36 24.41,108.36 24.23,108.53
  Top 0.406: AUDIO_CONN1.1 34.32,161.97
  Top 1.016: v40.79,133.2 40.79,154.99 34.32,161.46 AUDIO_CONN1.1
  Bottom 0.254: 20.3,108.28 v20.27,108.25
  Bottom 0.61: v24.35,108.28 20.3,108.28
  Bottom 1.016: v40.79,133.2 40.79,116.36 v22.1,97.66
  other vias: 22.56,98.09
  pour Top: 17.86,92.81 17.86,100.33 18.9,101.37 18.9,107.24 20.04,108.38 20.04,110.29 20.42,110.29 20.42,106.96 20.19,106.73 20.19,105.31 20.6,104.9 22.28,104.9 22.28,103.33 22.83,102.77 22.83,92.89 22.83,92.81
AVDD10  (via drill 0.3)
  Top 0.254: P3.8 64.93,73.5 65.63,72.8 v65.63,63.07
  Top 0.61: 68.15,37.85 R49.2 C53.2 R29.2 C55.2 69.8,41.96 | 68.15,37.85 C61.2 | v68.15,39.29 68.15,37.85 | 69.8,41.96 69.8,43.69 D7.1 | D9.- 69.85,41.91 69.8,41.96
  Bottom 0.254: v65.63,63.07 65.63,44.55 65.63,42.24 65.63,41.81 v68.15,39.29
BCLK
  Top 0.305: U11.13 23.52,117.47 R53.2
D+
  Top 0.254: U3.1 19.58,151.33 20.94,152.69 USB-TTL.A6 20.94,160.04 20.7,160.27 19.99,160.27 19.66,159.94 19.66,159.38 19.94,159.11 USB-TTL.B6
D-  (via drill 0.3)
  Top 0.254: U3.2 19.47,152.34 20.44,153.31 USB-TTL.A7 20.44,159.52 v20.32,159.64 | USB-TTL.B7 21.44,159.54 v21.57,159.66
  Bottom 0.254: v21.57,159.66 v20.32,159.64
DCLK  (via drill 0.3)  (1 unrouted)
  Top 0.254: FB1.2 C1.2 v23.8,71.7 | P3.14 v56.33,76.5
  Bottom 0.254: v23.8,71.7 51.54,71.7 v56.34,76.5
DIN
  Top 0.305: U11.14 22.87,118.35 R51.2
DTR  (via drill 0.3)
  Top 0.406: U3.4 v15.66,154.34 v15.67,154.33 | Q3.2 16.42,83.44 | 16.42,83.44 16.42,84.42 R26.2 | v14.58,83.14 16.13,83.14 16.42,83.44
  Bottom 0.406: v14.58,83.14 14.58,153.24 v15.67,154.33
GND  (via drill 0.3)
  Top 0.254: P3.51 60.35,92.86 59.99,92.5 P3.46 | P3.51 | v55.8,70.66 56.14,71 P3.3 59.96,71 60.35,70.61 P3.52 | 59.79,76 59.79,75.29 59.51,75 P3.11 55.04,75 C15.1 | 59.79,76 59.79,76.91 | 59.79,76.91 59.79,82.07 | 59.79,82.07 59.79,86.03 59.33,86.49 58.01,86.49 P3.34 P3.32 | P3.13 59.79,76 | 59.79,76.91 59.7,77 P3.15 P3.18 59.73,78.5 59.74,78.51 | 59.79,82.07 59.72,82 P3.25 P3.24 | P3.52
  Top 0.305: U11.19 19.62,116.73 18.87,117.47 18.87,117.85 C73.2
  other vias: 96.47,19.84 98.07,7.49 77.6,102.82 69.24,84.4 45.52,92.61 91.44,91.95 76.12,72.62 93.95,105.92 46.2,142.67 1.73,16.56 90.22,71.3 97.87,77.44 66.6,89.36 89.53,16.33 15.54,5.61 96.29,92.02 52.93,77.62 22.4,35.71 97.61,70.79 96.85,2.72 8.99,54.91 66.04,97.76 42.9,9.53 10.03,10.85 24.66,21.54 12.67,14.22 97.69,12.17 23.14,132.46 44.45,11.25 59.31,135.94 80.85,49.53 2.54,2.9 76.53,85.95 37.06,99.06 23.09,6.32 43.71,90.55 2.67,8.89 85.39,24.46 90.42,82.37 38.99,5.77 97.54,83.39 89.87,2.59 90.02,126.36 86.74,112.52 46.74,121.87 96.85,61.47 1.93,33.6 12.67,22.73 7.95,75.41 2.84,74.9 11.33,36.93 10.36,28.91 14.78,36.09 3.94,26.49 2.26,84.58 8.46,85.75 8.56,71.37 39.52,35.89 7.54,45.59 8,56.11 8.1,52.3 10.82,55.96 33.88,55.8 20.8,54.31 16.08,51.61 13.89,50.11 22,52.65 19.38,47.4 23.7,50.6 10.21,54.33 12.57,47.8 18.9,45.42 13.28,45.26 16.08,47.68 30.25,55.85 24.49,65.23 4.8,113.18 16.18,28.78 60.71,142.95 57.53,60.4 2.41,129.51 4.04,123.9 4.57,69.7 24.77,72.85 21.34,66.75 34.32,60.05 29.01,65.89 33.58,65.13 30.99,78.21 27.89,91.97 28.14,86.13 45.92,88.7 4.37,97.87 46.89,132.41 92.74,27.94 90.55,48.29 33.91,139.27 93.17,116.33 7.06,104.29 93.88,127.91 92.79,123.19 92.68,59.87 29.95,121.89 45.21,113 93.09,69.49 44.22,86.97 93.52,86.46 2.13,162.48 1.47,155.7 9.32,163.17 11.73,162.89 1.73,160.32 30.84,160.5 38.51,159.49 28.37,162.43 45.69,158.09 71.73,162.46 58.95,156.84 61.47,157.71 82.35,162.03 98.3,163.47 98.37,157.84 89.97,162.84 97.26,153.31 97.56,151 96.72,148.77 79.68,155.4 82.02,145.57 49.33,157.96 73.69,137.64 83.9,147.62 1.93,149.17 64.21,105.05 90.53,134.62 57.25,112.52 73.41,105.16 61.21,75.67 65.91,84.91 80.85,58.93 48.59,75.67 53.57,74.73 44.86,28.88 44.12,24.08 27.53,22.53 38.46,23.88 32.77,35.76 50.5,47.45 49.4,39.5 45.06,37.57 56.95,47.73 48.79,64.24 48.95,59.69 53.11,67.92 57.81,63.4 59.36,55.4 61.77,50.6 66.95,46.63 72.11,64.39 72.16,55.58 72.47,46.61 65.81,30.15 71.63,26.75 75.92,6.12 60.88,4.47 50.6,23.42 54.81,22.53 76.23,143.76 72.19,156.41 48.92,85.8 52.65,85.75 56.46,85.95 56.13,77.9 49.1,77.14 23.42,53.8 29.92,60.17 23.52,147.93 24.23,147.93 24.99,147.98 24.99,147.24 24.16,147.24 23.5,147.19 23.47,146.58 24.16,146.56 24.92,146.56 25.12,145.95 24.38,145.9 23.57,145.77 24.08,145.34 25.02,145.36 23.06,151.56 18.31,150.57 11.18,154.58 11.86,154.58 12.7,154.58 12.78,153.8 12.17,153.9 11.33,153.82 11.13,153.01 11.89,153.03 12.67,153.06 12.6,152.3 11.84,152.22 11.2,152.22 28.98,115.77 23.14,113.49 26.09,109.8 17.58,122.96 17.55,137.19 34.06,131.9 35.51,121.97 45.92,101.45 52.45,99.09 57,101.8 56.21,93.04 77.7,94.34 64.06,60.66 78.69,119.91 7.42,133.43 1.98,134.42 29.95,132.16 24.28,123.29 61.87,37.36 58.19,34.98 62.56,39.75 72.85,41.78 7.67,37.59 7.57,41.4 53.54,144.6 17.09,126.21
  pour Top (isolate 0.305, rank 6): -10,180 -10,-20 150,-20 150,180
  pour Bottom (isolate 0.305, rank 6): -5,-20 150,-20 150,180 -5,180
IO0  (via drill 0.3)
  Top 0.406: U1.27 24.05,59.56 23.5,59 v14.58,59 | BOOT.2 12.82,81.88 R22.1 Q3.3 | Q3.3 | Q3.3 14.58,81.67 v14.58,81.11
  Bottom 0.406: v14.58,81.11 v14.58,59
IO1  (via drill 0.3)
  Top 0.254: P3.39 60.99,89 61.38,88.6 v63.45,88.6
  Top 0.406: U1.39 8.81,58.75 10.03,57.53 21.85,57.53 v22.26,57.94
  Bottom 0.406: v63.45,88.6 63.45,62.61 58.78,57.94 v22.26,57.94
IO2  (via drill 0.3)
  Top 0.406: U1.38 10.08,59.36 11.18,58.27 v17.63,58.27 | R54.1 v26.31,120.95
  Bottom 0.406: v17.63,58.27 17.63,118.97 19.63,120.98 26.29,120.98 v26.31,120.95
IO3  (via drill 0.3)
  Top 0.406: R38.2 v28.83,143.03 R34.1 | U1.15 21.86,44.52 v21.84,44.5
  Bottom 0.406: v21.84,44.5 21.84,47.6 15.93,53.52 15.93,140.79 18.16,143.03 v28.83,143.03
IO4  (via drill 0.3)
  Top 0.254: U1.4 11.35,41.97 15.14,38.18 39.42,38.18 46.89,45.64 46.89,81.05 47.74,81.9 v53.75,81.9 | P3.31 53.95,85 v53.75,85.2
  Bottom 0.254: v53.75,81.9 v53.75,85.2
IO5
  Top 0.254: U1.5 12.62,41.79 15.65,38.76 39.19,38.76 46.3,45.87 46.3,81.28 47.52,82.5 P3.26
IO6
  Top 0.254: U1.6 13.89,41.56 16.13,39.32 38.81,39.32 45.72,46.23 45.72,81.51 47.21,83 P3.27
IO7
  Top 0.254: U1.7 15.16,41.35 16.64,39.88 38.58,39.88 45.19,46.48 45.19,81.81 46.87,83.5 P3.28
IO8
  Top 0.254: U1.12 21.51,42.07 22.05,41.53 37.64,41.53 43.41,47.3 43.41,82.53 47.88,87 P3.35
IO9
  Top 0.254: U1.17 25.31,47.07 40.21,47.07 41.53,48.39 41.53,83.06 46.97,88.5 P3.38
IO10  (via drill 0.3)
  Top 0.254: P3.21 48.61,80 48.39,79.78 v47.6,79.78 | U1.18 39.54,48.33 40.92,49.71 v40.92,79.78
  Bottom 0.254: v47.6,79.78 v40.92,79.78
IO11/MIDI_OUT
  Top 0.406: U1.19 31.15,49.59 R7.1
IO12/MIDI_IN
  Top 0.406: U1.20 38.98,50.87 40.23,52.12 40.23,89.2 44.65,93.62 44.65,94.28 | U7.4 44.65,94.28 | R9.2 44.68,94.26 44.65,94.28
IO13  (via drill 0.3)
  Top 0.254: P3.20 48.89,79.5 48.56,79.17 v48,79.17 | U1.21 25.31,52.15 38.51,52.15 39.55,53.19 v39.55,79.17
  Bottom 0.254: v48,79.17 v39.55,79.17
IO14  (via drill 0.3)
  Top 0.254: P3.23 v47.8,81 | U1.22 37.84,53.41 38.93,54.5 v38.93,81
  Bottom 0.254: v47.8,81 v38.93,81
IO15
  Top 0.254: U1.8 16.43,41.43 17.45,40.41 38.3,40.41 44.6,46.71 44.6,82.07 46.53,84 P3.29
IO16
  Top 0.254: U1.9 17.7,42.09 18.82,40.97 37.97,40.97 44.02,47.02 44.02,82.35 46.17,84.5 P3.30
IO17/I2C_SDA  (via drill 0.3)
  Top 0.406: P4.5 v56.99,16 52.02,16 49.52,18.5 P1.5 22.89,18.49 v21.77,17.37 21.22,16.83 J2.2 | v56.16,34.42 56.16,33.44 R47.1 | v19.15,41.76 19.15,42.57 U1.10
  Bottom 0.406: v56.99,16 56.99,33.59 v56.16,34.42 | v19.15,41.76 19.15,19.99 v21.77,17.37
IO18/I2C_SCL  (via drill 0.3)  (1 unrouted)
  Top 0.406: P4.4 51.37,15 48.87,17.5 P1.4 24.36,17.5 24.08,17.22 v24,17.14 23.22,16.36 J2.1 | R42.1 51.57,31.93 R27.1 v48.72,31.93 | v20.04,41.76 20.04,42.55 U1.11
  Bottom 0.406: v48.72,17.5 v48.72,31.93 | v20.04,41.76 20.04,21.11 v24,17.14
IO19  (via drill 0.3)
  Top 0.305: 92.25,153.75 R20.2 | U1.13
  Top 0.406: 92.25,153.75 92.25,149.17 62.43,119.36 62.05,118.97 v26.31,118.97 25.78,118.97 R51.1 | v22.99,43.74 22.99,42.96 U1.13
  Bottom 0.406: v22.99,43.74 22.99,47.68 18.39,52.27 18.39,117.88 19.48,118.97 v26.31,118.97
IO20  (via drill 0.3)
  Top 0.305: U1.14
  Top 0.406: v93.07,150.14 93.07,148.59 63.61,119.14 62.69,118.21 v26.31,118.21 25.78,118.21 R53.1 | v91.44,150.14 91.44,153.03 R21.2 | v23.82,43.74 23.82,42.98 U1.14
  Bottom 0.406: v93.07,150.14 v91.44,150.14 | v23.82,43.74 23.82,48.18 19.15,52.86 19.15,117.42 19.94,118.21 v26.31,118.21
IO21  (via drill 0.3)
  Top 0.254: P3.22 48.22,80.5 v48.12,80.4 | v38.33,80.4 38.33,55.17 37.85,54.69 25.31,54.69 U1.23
  Bottom 0.254: v38.33,80.4 v48.12,80.4
IO38  (via drill 0.3)
  Top 0.254: P3.36 47.57,87.5 42.77,82.7 v42.77,61.7 | U1.31 18.97,61.13 19.53,61.7 v25.83,61.7
  Bottom 0.254: v25.83,61.7 v42.77,61.7
IO39  (via drill 0.3)
  Top 0.254: R40.1 P3.40 v61.7,89.5
  Top 0.305: U1.32 17.7,66.39 20.52,69.22 v22,69.22
  Bottom 0.254: v22,69.22 52.22,69.22 61.7,78.69 v61.7,89.5
IO40  (via drill 0.3)
  Top 0.254: P3.42 59.46,90.5 59.79,90.83 v60.94,90.83
  Top 0.305: U1.33 16.43,66.24 20.12,69.93 v22.5,69.93
  Bottom 0.254: v22.5,69.93 51.84,69.93 60.94,79.02 v60.94,90.83
IO41  (via drill 0.3)
  Top 0.254: R45.1 54.35,90 P3.41 60.12,90 v60.27,90.15
  Top 0.305: U1.34 15.16,66.09 19.74,70.66 v22,70.66
  Bottom 0.254: v22,70.66 51.51,70.66 60.27,79.43 v60.27,90.15
IO42
  Top 0.305: U1.35 13.89,66 FB1.1
IO45  (via drill 0.3)
  Top 0.254: P3.19 49.15,78.99 47.5,77.34 v47.5,58.7
  Top 0.305: v26.3,58.7 25.52,58.7 U1.26
  Top 0.406: U1.26 24.2,58.48 22.45,56.74 v14.58,56.74 | v11.02,39.19 R4.2
  Bottom 0.254: v26.3,58.7 v47.5,58.7
  Bottom 0.406: v11.02,39.19 11.02,50.11 14.58,53.67 v14.58,56.74
IO46
  Top 0.254: U1.16 39.82,45.78 42.14,48.11 42.14,82.83 47.31,88 P3.37
IO47  (via drill 0.3)
  Top 0.406: v15.24,55.93 25.29,55.93 U1.24 | R59.2 15.24,148.97 v15.24,149.56
  Bottom 0.406: v15.24,55.93 v15.24,149.56
IO48  (via drill 0.3)
  Top 0.406: v67.13,33.73 R41.2 | v26.3,57.2 26.29,57.22 U1.25
  Bottom 0.406: v26.3,57.2 61.37,57.2 64.64,53.92 64.64,36.22 v67.13,33.73
LCD_RST
  Top 0.254: P3.7 C15.2 R1.1
LED+  (via drill 0.3)
  Top 0.254: P3.49 P3.50 58.22,94.25
  Top 0.406: v58.9,125.8 20.47,125.8 20.02,125.8 19.11,125.8 v16.61,128.29 C11.2 D1.- 14.75,132.23 C12.2 | U2.5 15.85,139.55 16.05,139.75 v16.61,139.75
  Top 0.61: 58.22,94.25 v58.9,94.25
  Bottom 0.406: v58.9,94.25 v58.9,125.8 | v16.61,128.29 v16.61,139.75
LED-  (via drill 0.3)
  Top 0.254: 58.27,93.27 P3.47 P3.48
  Top 0.406: v59.61,126.5 20.85,126.5 20.6,126.5 19.7,126.5 16.79,129.41 R33.2 R32.2 16.8,133.46 U2.3
  Top 0.61: 58.27,93.27 v59.61,93.27
  Bottom 0.406: v59.61,93.27 v59.61,126.5
LOUT  (via drill 0.3)
  Top 1.016: AUDIO_CONN1.2 38.42,149.2 AUDIO_CONN1.4 38.57,133.18 v38.58,133.17 | R68.1 23.9,103.83 v23.9,103.07 23.9,102.17 C84.1
  Bottom 1.016: v38.58,133.17 38.58,117.75 v23.9,103.07
LRC
  Top 0.305: U11.15 22.22,119.32 R54.2
N$1
  Top 0.61: D6.1 C47.2 R11.1
N$2
  Top 0.406: R26.1 16.2,86.16 16.2,87.13 Q4.1
N$3
  Top 0.406: Q3.1 17.36,80.91 18.77,82.32 R25.1
N$4
  Top 0.61: R52.1 R50.2 R49.1 C61.1
N$5
  Top 0.254: P3.4 54.58,71.5 R66.2 R65.1
N$6
  Top 0.254: USB-NATIVE.A5 91.83,157.29 R15.2
N$7
  Top 0.406: PWR.C R19.2
N$8
  Top 0.61: C48.2 D6.3
N$9
  Top 0.61: U4.1 59.75,36.41 59.46,36.7 59.46,41.02 | 59.46,41.02 59.46,41.81 L2.P$2 | 59.46,41.02 59.51,41.07 C48.1 C49.2 66.75,41.07 D9.+
N$10
  Top 0.254: USB-TTL.A5 21.94,155.74 R13.2
N$11
  Top 0.254: USB-TTL.B5 18.94,155.82 R12.2
N$12
  Top 0.61: C49.1 65.86,42.81 D7.3
N$13
  Top 0.61: R18.2 C50.2 D7.2
N$14
  Top 0.254: USB-NATIVE.B5 88.83,155.64 R14.2
N$15
  Top 0.61: U4.3 63.06,38.31 R52.2
N$16
  Top 0.61: R30.2 R3.1 74.64,36.78 RW1.2 77.13,36.54 RW1.3
N$17
  Top 0.406: L1.P$2 14.61,136.3 U2.1 14.88,136 D1.+ 14.4,134.01 R23.2
  pour Top: 8.59,135.23 12.32,135.23 12.85,134.7 12.85,133.68 15.11,133.68 15.11,136.8 8.59,136.8
N$18
  Top 0.406: R35.1 59.94,33.4 Q1.3
N$19
  Top 0.61: U4.4 56.29,38.31 R64.1
N$20
  Top 0.406: Q1.1 64.51,31.38 R43.2 R41.1
N$22
  Top 0.406: C2.2 R23.1
N$23  (via drill 0.3)
  Top 0.813: R5.2 v53.03,108.15 | MIDI_IN_CONN2.3 55.65,142.61 v53.03,140
  Top 1.016: MIDI_IN_CONN2.3 MIDI_IN_CONN2.5
  Bottom 0.813: v53.03,108.15 v53.03,140
N$24
  Top 0.406: U2.4 17.3,139.11 17.3,140.08 16.59,140.79 R39.1 R31.2 16.46,143.26 Q7.3
N$26
  Top 0.813: R5.1 D4.- 49.73,107.35 U7.1
N$27  (via drill 0.3)
  Top 0.813: v54.71,94.26 R6.2 | MIDI_OUT_CONN3.3 68.98,140.53 68.99,140.53 68.99,138.71 61.08,130.8 v54.71,130.8
  Top 1.016: MIDI_OUT_CONN3.3 MIDI_OUT_CONN3.5
  Bottom 0.813: v54.71,94.26 v54.71,130.8
N$29
  Top 0.406: Q7.1 16.85,147.33 R60.2 R59.1
N$30
  Top 0.406: U6.2 20.07,147.4 R28.1
N$31
  Top 0.406: U6.7 R61.2
N$32
  Top 0.406: U6.6 29.01,146.13 R62.2
N$33
  Top 0.406: CHRG.C 29.54,149 30.79,147.75 R61.1
N$34
  Top 0.406: R62.1 31.77,146.81 31.77,148.89 DONE.C
N$35  (via drill 0.3)
  Top 0.406: 32.64,49.63 R7.2
  Top 0.813: v37.41,82 v37.41,55.57 | R7.2 v37.41,49.58 | MIDI_OUT_CONN3.4 66.23,140.25 58.95,132.97 v50.04,132.97
  Top 1.016: MIDI_OUT_CONN3.2 66.08,149.2 MIDI_OUT_CONN3.4
  Bottom 0.813: v37.41,55.57 v37.41,49.58 | v37.41,82 50.04,94.62 v50.04,132.97
N$36  (via drill 0.3)
  Top 0.406: D4.+
  Top 0.813: 51.92,149.99 51.92,148.39 51.46,147.93 | U7.2 47.19,107.45 D4.+ 47.21,108.25 47.93,108.97 v51.46,108.97 | v51.46,142 51.46,147.93 | 51.46,147.93 51.46,150.64 51.05,151.05
  Top 1.016: MIDI_IN_CONN2.2 48.8,153.3 51.05,151.05 MIDI_IN_CONN2.4
  Bottom 0.813: v51.46,108.97 v51.46,142
N$43
  Top 0.305: U11.18 20.27,117.82 C73.1
  Top 1.016: C73.1 20.53,122.18 C79.+
N$44
  Top 0.305: U11.7 22.87,107.99 23.52,107.34 24.55,107.34 R67.2
N$45
  Top 0.305: U11.4 20.92,110.63 21.69,111.4 26.93,111.4 C77.1
N$46
  Top 0.406: U3.9 7.38,152.34 R17.2
N$47
  Top 0.305: U11.2 19.62,110.58 21.13,112.09 25.17,112.09 26.52,113.44 27.07,113.44 C77.2
N$49
  Top 0.406: U3.8 R2.2
N$76
  Top 0.61: U5.4 11.24,146.42 C45.1
OUTL
  Top 0.305: U11.6 22.22,107.51 R68.2
RESET  (via drill 0.3)
  Top 0.406: v10.08,44.15 U1.3 | RST.2 4.08,88.39 C8.1 Q4.3 13.89,88.36 v13.89,86.82 13.89,86.36 R16.1
  Bottom 0.406: v10.08,44.15 10.08,50.29 13.89,54.1 v13.89,86.82
ROUT  (via drill 0.3)
  Top 0.406: R67.1
  Top 1.016: AUDIO_CONN1.5 AUDIO_CONN1.3 42.55,159.47 v42.55,133.22 | C83.1 v26.36,99.47 25.81,100.03 25.81,100.64 | R67.1 25.81,100.64 | 24.79,99.54 24.79,99.62 25.81,100.64
  Bottom 1.016: v42.55,133.22 42.55,115.65 v26.36,99.47
RTS  (via drill 0.3)
  Top 0.406: v9.3,155.96 9.29,155.95 U3.6 | R25.2 18.77,87.37 16.98,89.17 16.82,89.33 | 16.82,89.33 Q4.2 | v13.89,89.75 16.4,89.75 16.82,89.33
  Bottom 0.406: v13.89,89.75 13.89,146.74 9.3,151.33 v9.3,155.96
RXD/IO44  (via drill 0.3)
  Top 0.406: v4.32,153.34 R2.1 | U1.36 12.62,61.34 v12.04,61.92
  Bottom 0.406: v12.04,61.92 12.04,145.62 v4.32,153.34
TP_INT  (via drill 0.3)
  Top 0.406: P4.2 v56.19,13 50.42,13 47.92,15.5 P1.2 | R36.1 R37.1 v56.19,27.74
  Bottom 0.406: v56.19,27.74 v56.19,13
TP_RST  (via drill 0.3)
  Top 0.406: 58.34,14 P4.3 | R44.1 57.79,31.9 | 57.79,31.9 C13.2 | 57.79,31.9 v57.79,31.14 v57.78,31.14 | v57.78,13.99 58.34,13.99 58.34,14 | 57.79,31.9 57.79,33.38 R35.2 | 58.34,14 50.9,14 48.4,16.5 P1.3
  Bottom 0.406: v57.78,31.14 v57.78,13.99
TXD/IO43  (via drill 0.3)
  Top 0.406: v4.57,151.76 R17.1 | U1.37 v11.35,61.26 v11.35,61.27
  Bottom 0.406: v11.35,61.27 11.35,144.98 v4.57,151.76
USB_D+
  Top 0.254: USB-NATIVE.A6 90.83,157.3 | 90.83,157.3 90.83,155.38 R21.1 | USB-NATIVE.B6 89.83,157.56 90.04,157.35 90.5,157.35 | 90.5,157.35 90.78,157.35 90.83,157.3 | 90.83,156.97 90.83,157.02 90.5,157.35 | 90.5,157.35 90.83,157.68 90.83,157.71
USB_D-
  Top 0.254: R20.1 91.33,156.24 USB-NATIVE.B7 91.33,159.24 91.08,159.49 90.53,159.49 90.33,159.29 USB-NATIVE.A7
VBAT
  Top 0.406: BAT.+ 26.43,139.79 C44.1 | C44.1 C40.1 26.49,142.32 | 26.49,142.32 R34.2 26.49,143.94 U6.5 | Q6.3 26.47,142.34 26.49,142.32 | D11.+ 26.36,139.72 C44.1
  pour Top: 26.97,134.62 25.65,134.62 24,136.27 24,142.85 26.21,145.06 28.07,145.06 28.07,144.48 27.05,143.46 27.05,134.7
VBUS  (via drill 0.3)
  Top 0.254: USB-TTL.VBUS2 18.24,157.15 v18.21,157.12
  Top 0.61: USB-TTL.VBUS2 18.24,156.72 C7.2 | USB-TTL.VBUS1 23.14,157.68 v23.14,157.12 23.14,156.54 23.39,156.29 23.44,156.29 | 23.44,156.29 25.04,156.29 | 25.04,156.29 27.06,156.29 D10.A | C4.2 23.39,156.24 23.44,156.29 | C6.2 24.89,156.13 25.04,156.29
  Bottom 0.61: v18.21,157.12 v23.14,157.12
VCOM  (via drill 0.3)
  Top 0.254: VCOM.T 74.88,70.97 v74.88,71.98 74.88,87.76 70.64,92 P3.45 | P3.5 64.68,72 v64.69,71.98
  Top 0.61: R29.1 73,38.33 R3.2 74.64,38.3 RW1.1 C52.2 VCOM.T
  Bottom 0.254: v64.69,71.98 v74.88,71.98
VGH
  Top 0.254: P3.10 65.56,74.5 68.68,71.37 VGH.T
  Top 0.61: R18.1 R24.2 C51.2 68.45,53.98 | 68.45,53.98 C56.2 C57.2 68.45,58.98 VGH.T | D8.C 68.47,53.96 68.45,53.98
VGL
  Top 0.254: P3.9 65.24,74 66.67,72.57 VGL.T
  Top 0.61: R11.2 C46.2 R10.2 66.65,53.92 | 66.65,53.92 66.65,55.52 C58.2 C59.2 66.7,59.11 VGL.T | D5.A 66.65,53.92
VNEG
  Top 0.305: U11.5 21.57,106.14 C78.1
VOUT  (via drill 0.3)
  Top 0.406: Q6.2 22.34,139.75 D11.- 22.37,138.89 | 22.37,138.89 22.37,137.58 D3.C | D2.C 22.33,138.84 22.37,138.89
  Top 0.813: 21.67,137.03 21.67,137.14 D2.C 20.52,138.28 v20.52,137.41 | v5.4,142.26 SW1.2 SW1.2@1 | v20.52,124.8 v5.4,124.8
  Bottom 0.813: v20.52,137.41 v20.52,124.8 | v5.4,124.8 v5.4,142.26
  pour Top: 18.87,136.53 22.73,136.53 22.73,141.6 21.89,141.6 21.89,140.74 21.16,140 18.87,140
VPWR
  Top 0.254: SW1.3 3.84,139.86 3.94,139.95
  Top 0.406: U2.6 14.9,139.95 | 14.9,139.95 14.9,140.76 R39.2 | L1.P$1 11.53,140 | 11.53,140 12.8,140 | 12.8,140 14.85,140 14.9,139.95 | C43.2 12.9,140.1 12.8,140 | U5.3 11.24,140.29 11.53,140 | U5.1 9.34,139.96 9.35,139.95 | C41.1 7.87,140.06 7.98,139.95
  Top 0.61: SW1.3@1 1.43,139.95 3.94,139.95 6.66,139.95 | 6.66,139.95 VPWR.T | 6.66,139.95 7.98,139.95 9.35,139.95 10.62,139.95 L1.P$1
  pour Top: 15.16,138.07 15.16,141.22 14.15,141.22 13.46,141.91 13.46,142.85 11.02,142.85 11.02,141.4 10.82,141.2 9.86,141.2 9.63,141.43 9.55,141.5 9.55,142.85 7.39,142.85 7.39,141.81 6.38,140.79 0.56,140.79 0.56,139.85 0.56,139.8 0.56,139.78 13.46,139.78 14.17,139.06 14.17,138.1 14.17,138.07

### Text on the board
tPlace: CHRG | C36 | C41 | + | - | + | - | 18650 battery 19*37*67 Section 2 | tulip.computer | Tulip Creative Computer v4r10 | GND | +3V3 | IO17/SDA | IO18/SCL
tNames: U4
tValues: Close
Measures: Units: Inches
